(* Logix 5000 AddOnInstructionDefinition export Banner_Q2X_Param_v4; software revision 33.00 *)

TYPE Banner_IOL_Port_v4 :   // UDT that has all of the data items necessary to communicate with a specific Port on a IO-Link Master
STRUCT
   Port_Controlled : INT;   // Each bit represents a port on an IO-Link Master. Set to 1 to tell AOI to control that port.
   Port_Activate : INT;   // Each bit represents a port on an IO-Link Master. When ON that port will process any commands in queue.
   Port_Read : INT;   // Each bit represents a port on an IO-Link Master. Used to determine when device AOI has requested a Read command.
   Port_Write : INT;   // Each bit represents a port on an IO-Link Master. Used to determine when device AOI has requested a Write command.
   Port_RW_Complete : INT;   // Each bit represents a port on an IO-Link Master. Tells device AOI that Read or Write request has been completed.
   Port_Device_Read : INT;
   Data_Transfer : SINT[190];   // Array to transfer data from IO-Master to device AOIs.
END_STRUCT
END_TYPE

TYPE Banner_Q2X_BDC_v4 :   // All of the BDC data for channels 1 and 2.
STRUCT
   SP1 : DINT;   // Switchpoint.
   SP2 : DINT;   // In 2pt window mode, defines the second switching point. In other modes, SP2 is unused and must be 0.
   Switchpoint_Logic : SINT;   // 0 = Light operate, 1 = Dark operate
   BDC_Mode : SINT;   // 1 = 1pt Object Set, 128 = 2pt static BGS, 129 = 2pt Window FGS, 130 = 1pt Window FGS, 131 = Dual Mode.
   Hysteresis : INT;   // A value of 0 will result in automatically calculated hysteresis.
   Delay_Mode : SINT;   // 0 = Disabled, 1 = On Off Delay, 2 = Oneshot.
   Delay_Timer_1 : DINT;   // 0 to 90000. On delay and oneshot time.
   Delay_Timer_2 : DINT;   // 0 to 90000. Off delay only.
   Teach_Offset : SINT;   // 0 = Auto, 1 = User Selected
   FGS_Window_Size : SINT;   // 0 = Auto, 1 = User Selected
   User_Teach_Offset : DINT;   // In Object Set or Window (FGS) mode this value can be either positive or negative. In all other modes must be zero.
   FGS_User_Window_Size : DINT;   // Mode must be Window FGS. Set the +/- window value. If FGS Window Size is set to Auto this value must to set to zero.
   Auto_Thresholding : SINT;   // 0 = Slow, 1 = Medium, 2 = Fast, 3 = Off.
END_STRUCT
END_TYPE

TYPE Banner_Q2X_Pulse_Freq_v4 :
STRUCT
   Near_Freq : DINT;   // 1 to 100000 in Hz
   Far_Freq : DINT;   // 1 to 100000 in Hz
   SP1 : DINT;   // Switchpoint
   SP2 : DINT;   // In 2pt Window FGS teach, define the second switching point. In other modes SP2 should be zero.
   Pulse_Freq_LOS : DINT;   // Default value of 50. This is the Hz that the units outputs when a Loss of Signal occurs.
END_STRUCT
END_TYPE

TYPE Banner_Q2X_RD_v4 :   // UDT that stores the Write Data for a Q2X.
STRUCT
   Master_Cycle_Time : INT;
   Min_Cycle_Time : INT;
   M_Sequence_Capability : INT;
   IO_Link_Version_ID : INT;
   Process_Data_Input_Length : INT;
   Process_Data_Output_Length : INT;
   Combined_Vendor_ID : DINT;   // IO-Link Vendor ID
   Vendor_ID1 : INT;
   Vendor_ID2 : INT;
   Combined_Device_ID : DINT;   // IO-Link Device ID
   Device_ID1 : INT;
   Device_ID2 : INT;
   Device_ID3 : INT;
   Serial_Number : STRING;
   Teach_State : SINT;
   SP1_TP1 : SINT;
   SP1_TP2 : SINT;
   Measurement_1 : DINT;
   Excess_Gain : DINT;   // Amount of singla measured over the minimum threshold.
   Stability : SINT;
   Emitter_Status : SINT;   // 0 = Active, 1 = Inactive
   Temperature : DINT;
   Last_Taught_Temperature : DINT;   // Internal Temperature the last time device was taught.
   MDC_Lower_Limit : DINT;
   MDC_Upper_Limit : DINT;
   MDC_Unit : INT;
   MDC_Scale : SINT;
END_STRUCT
END_TYPE

TYPE Banner_Q2X_v4 :   // All of the parameters for a Q2X.
STRUCT
   Initial_Global_Read : BOOL;   // Determines if all of the IO-Link data has been read into the PLC yet
   Command : INT;   // Value placed in here will activate a read or write to a specifc IO-Link Index
   Read : Banner_Q2X_RD_v4;   // Read Only Data
   Write : Banner_Q2X_WD_v4;   // Write Data
   Archive : Banner_Q2X_WD_v4;   // Archive Data
   Reset : BOOL;   // Resets AOI. This will force a complete parameter read of the sensor.
END_STRUCT
END_TYPE

TYPE Banner_Q2X_WD_v4 :   // UDT that stores the Write Data for a Q2X.
STRUCT
   System_Command : INT;   // See IODD file for list of commands that can be activated via the System Command interface
   Parameter_Access_Lock : SINT;   // Write access to all parameters is prohibited while value is 1. Only this parameter can be adjusted when value is 1.
   Data_Storage_Lock : SINT;   // Automatic data storage is disabled when this value is equal to 1. Read access is not affected.
   Local_Parameterization_Lock : SINT;   // Parameterization via local control elements on device is disabled.
   Local_User_Interface_Lock : SINT;   // Operation of local user interface is disabled.
   Teach_in_Channel : SINT;   // 0 = Default, 1 = BDC1, 2 = BDC2
   Response_Speed : SINT;   // 0 = Speed 0, 1 = Speed 1, 2 = Speed 2, 3 = Speed 3
   Secondary_Output_Mode : SINT;   // 0 = Independent Output, 1 = Complementary Output, 2 = Pulse Frequency Output
   IOL_Filter_Time : INT;   // Time to average IOl process data measurement between updates
   Include_Binary : SINT;   // 0 = Include, 1 = Don't Include, 2= Measurement Device
   Measurement_1 : SINT;   // 0 = Disabled, 1 = Excess Gain, 2 = Excess Gain / 10, 3 = Channel 1 Dual Mode Percent
   Measurement_2 : SINT;   // 0 = Disabled, 1 = Distance Value, 2 = Displayed Distance, 3 = Channel 2 Dual Mode Percent
   BDC : Banner_Q2X_BDC_v4[3];
   Pulse_Freq : Banner_Q2X_Pulse_Freq_v4;
END_STRUCT
END_TYPE

ADD_ON_INSTRUCTION Banner_Q2X_Param_v4   (* revision 4.0, vendor Banner Engineering *)
// AOI to read and write parameter data to an IO-Link Q2X.
VAR_IN_OUT
   Q2X : Banner_Q2X_v4; {required}
   Port_Data : Banner_IOL_Port_v4; {required}
END_VAR
VAR_INPUT
   Port : DINT; {required}
END_VAR
VAR
   Local_Control : DINT; {access None}
   Global_Read_Command_Value : INT; {access None}
   Global_Write_Command_Value : INT; {access None}
   Command_Being_Processed : BOOL; {access None}
   Update_Archive : BOOL; {access None}
   Index_Write_Inprocess : INT; {access None}
   Index_Write_Control : INT; {access None}
   Inprocess_Index : DINT; {access None}
END_VAR

ROUTINE Logic   (* ladder *)
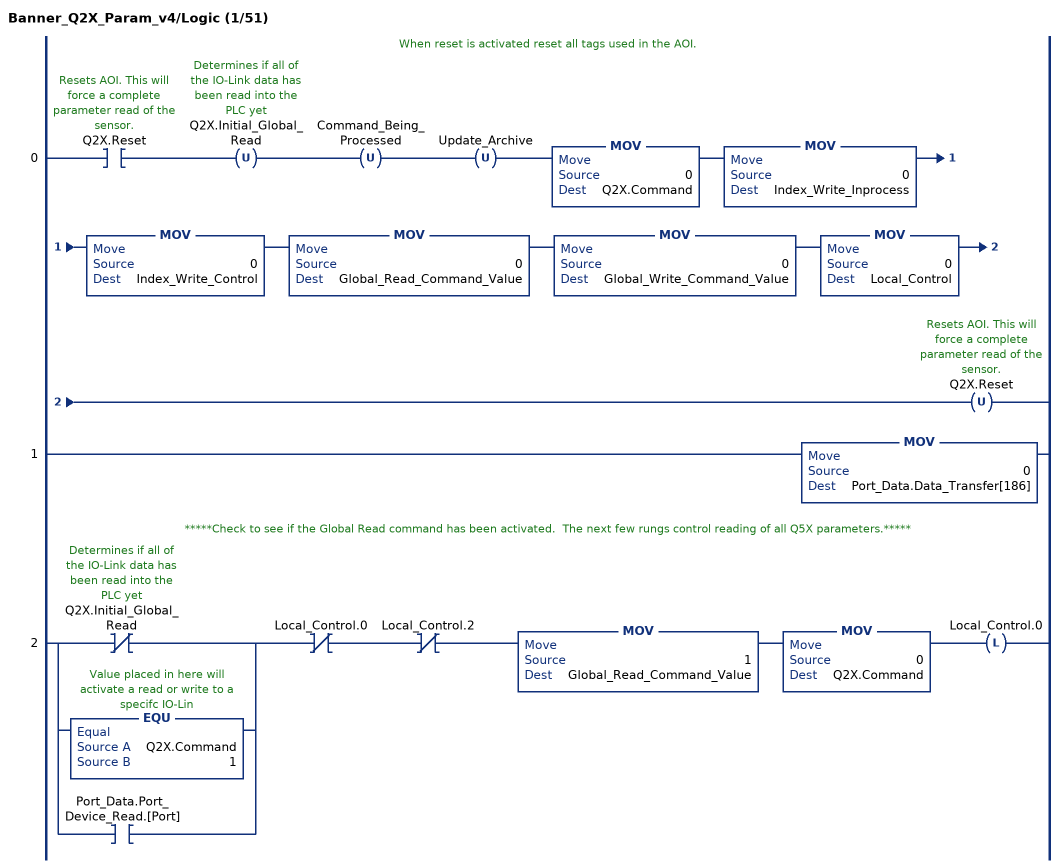
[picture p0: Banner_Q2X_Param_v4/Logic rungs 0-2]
   // When reset is activated reset all tags used in the AOI.
   0: XIC(Q2X.Reset)OTU(Q2X.Initial_Global_Read)OTU(Command_Being_Processed)OTU(Update_Archive)MOV(0,Q2X.Command)MOV(0,Index_Write_Inprocess)MOV(0,Index_Write_Control)MOV(0,Global_Read_Command_Value)MOV(0,Global_Write_Command_Value)MOV(0,Local_Control)OTU(Q2X.Reset);
   1: MOV(0,Port_Data.Data_Transfer[186]);
   // *****Check to see if the Global Read command has been activated.  The next few rungs control reading of all Q5X parameters.*****
   2: [XIO(Q2X.Initial_Global_Read) ,EQU(Q2X.Command,1) ,XIC(Port_Data.Port_Device_Read.[Port]) ]XIO(Local_Control.0)XIO(Local_Control.2)MOV(1,Global_Read_Command_Value)MOV(0,Q2X.Command)OTL(Local_Control.0);
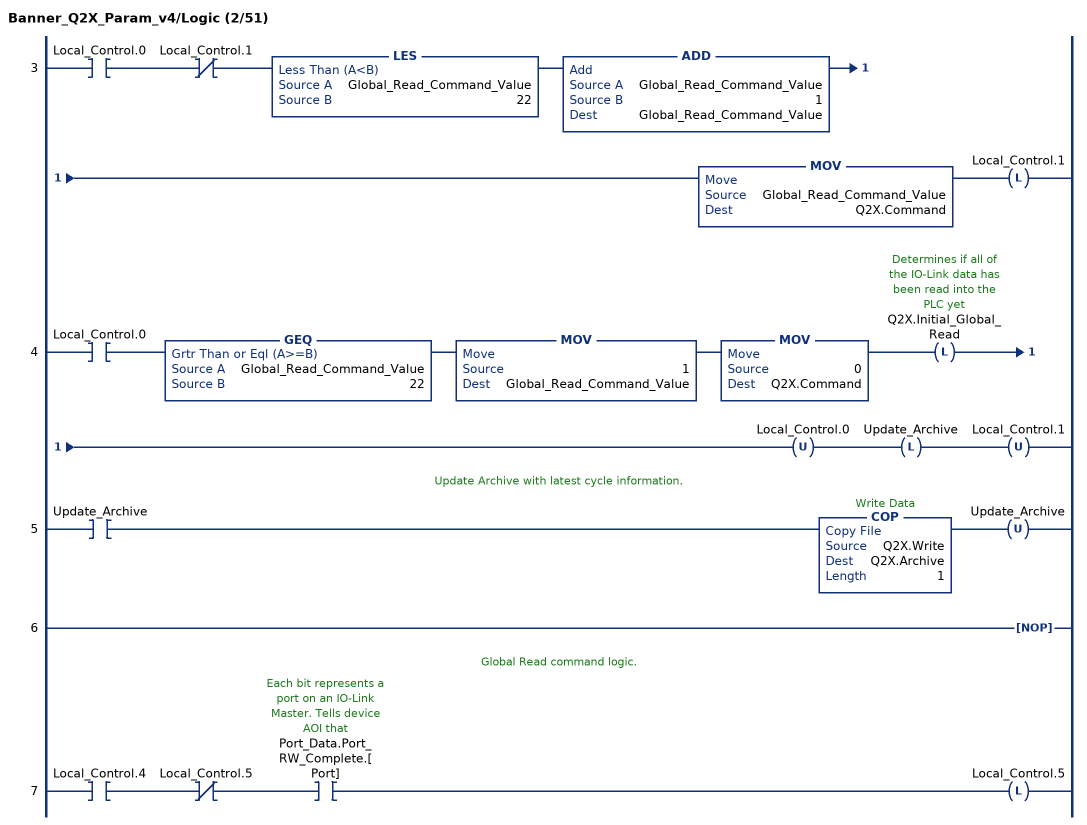
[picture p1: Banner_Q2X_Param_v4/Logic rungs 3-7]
   3: XIC(Local_Control.0)XIO(Local_Control.1)LES(Global_Read_Command_Value,22)ADD(Global_Read_Command_Value,1,Global_Read_Command_Value)MOV(Global_Read_Command_Value,Q2X.Command)OTL(Local_Control.1);
   4: XIC(Local_Control.0)GEQ(Global_Read_Command_Value,22)MOV(1,Global_Read_Command_Value)MOV(0,Q2X.Command)OTL(Q2X.Initial_Global_Read)OTU(Local_Control.0)OTL(Update_Archive)OTU(Local_Control.1);
   // Update Archive with latest cycle information.
   5: XIC(Update_Archive)COP(Q2X.Write,Q2X.Archive,1)OTU(Update_Archive);
   6: NOP();
   // Global Read command logic.
   7: XIC(Local_Control.4)XIO(Local_Control.5)XIC(Port_Data.Port_RW_Complete.[Port])OTL(Local_Control.5);
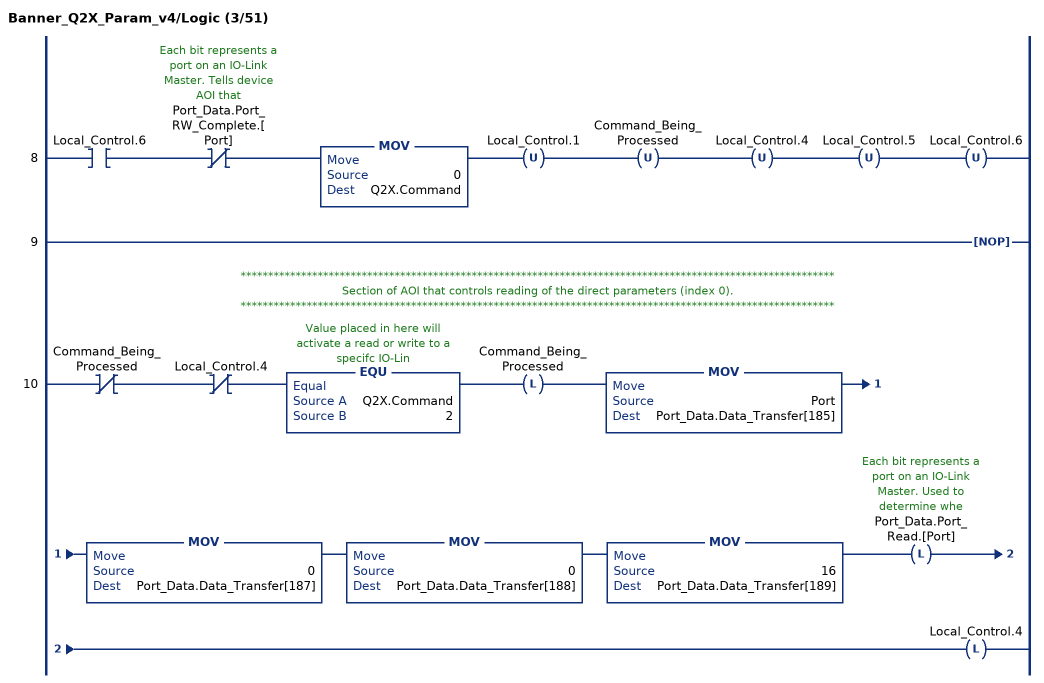
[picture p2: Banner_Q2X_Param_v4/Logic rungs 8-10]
   8: XIC(Local_Control.6)XIO(Port_Data.Port_RW_Complete.[Port])MOV(0,Q2X.Command)OTU(Local_Control.1)OTU(Command_Being_Processed)OTU(Local_Control.4)OTU(Local_Control.5)OTU(Local_Control.6);
   9: NOP();
   // ************************************************************************************************************
   // Section of AOI that controls reading of the direct parameters (index 0).
   // ************************************************************************************************************
   10: XIO(Command_Being_Processed)XIO(Local_Control.4)EQU(Q2X.Command,2)OTL(Command_Being_Processed)MOV(Port,Port_Data.Data_Transfer[185])MOV(0,Port_Data.Data_Transfer[187])MOV(0,Port_Data.Data_Transfer[188])MOV(16,Port_Data.Data_Transfer[189])OTL(Port_Data.Port_Read.[Port])OTL(Local_Control.4);
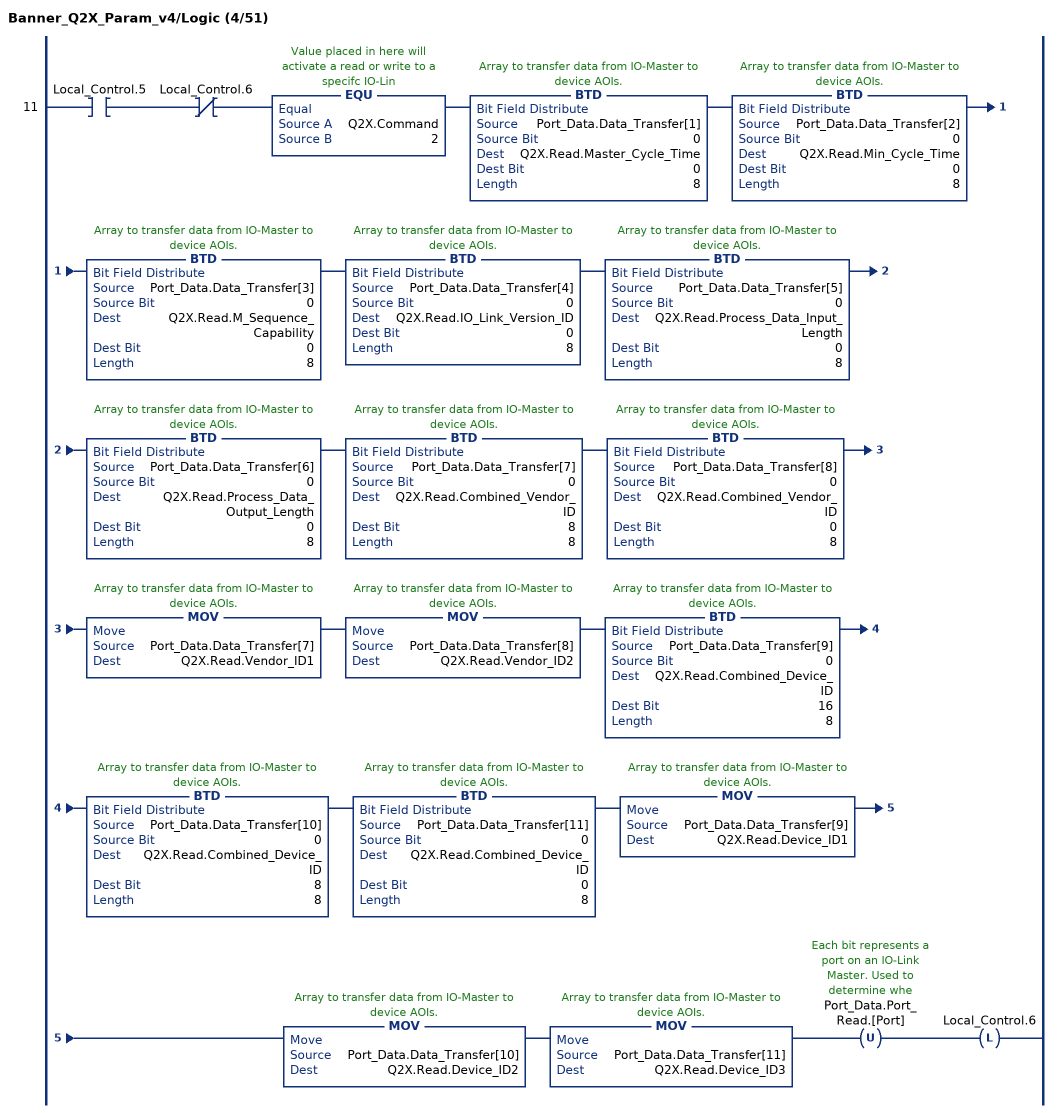
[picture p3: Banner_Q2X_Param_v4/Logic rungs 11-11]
   11: XIC(Local_Control.5)XIO(Local_Control.6)EQU(Q2X.Command,2)BTD(Port_Data.Data_Transfer[1],0,Q2X.Read.Master_Cycle_Time,0,8)BTD(Port_Data.Data_Transfer[2],0,Q2X.Read.Min_Cycle_Time,0,8)BTD(Port_Data.Data_Transfer[3],0,Q2X.Read.M_Sequence_Capability,0,8)BTD(Port_Data.Data_Transfer[4],0,Q2X.Read.IO_Link_Version_ID,0,8)BTD(Port_Data.Data_Transfer[5],0,Q2X.Read.Process_Data_Input_Length,0,8)BTD(Port_Data.Data_Transfer[6],0,Q2X.Read.Process_Data_Output_Length,0,8)BTD(Port_Data.Data_Transfer[7],0,Q2X.Read.Combined_Vendor_ID,8,8)BTD(Port_Data.Data_Transfer[8],0,Q2X.Read.Combined_Vendor_ID,0,8)MOV(Port_Data.Data_Transfer[7],Q2X.Read.Vendor_ID1)MOV(Port_Data.Data_Transfer[8],Q2X.Read.Vendor_ID2)BTD(Port_Data.Data_Transfer[9],0,Q2X.Read.Combined_Device_ID,16,8)BTD(Port_Data.Data_Transfer[10],0,Q2X.Read.Combined_Device_ID,8,8)BTD(Port_Data.Data_Transfer[11],0,Q2X.Read.Combined_Device_ID,0,8)MOV(Port_Data.Data_Transfer[9],Q2X.Read.Device_ID1)MOV(Port_Data.Data_Transfer[10],Q2X.Read.Device_ID2)MOV(Port_Data.Data_Transfer[11],Q2X.Read.Device_ID3)OTU(Port_Data.Port_Read.[Port])OTL(Local_Control.6);
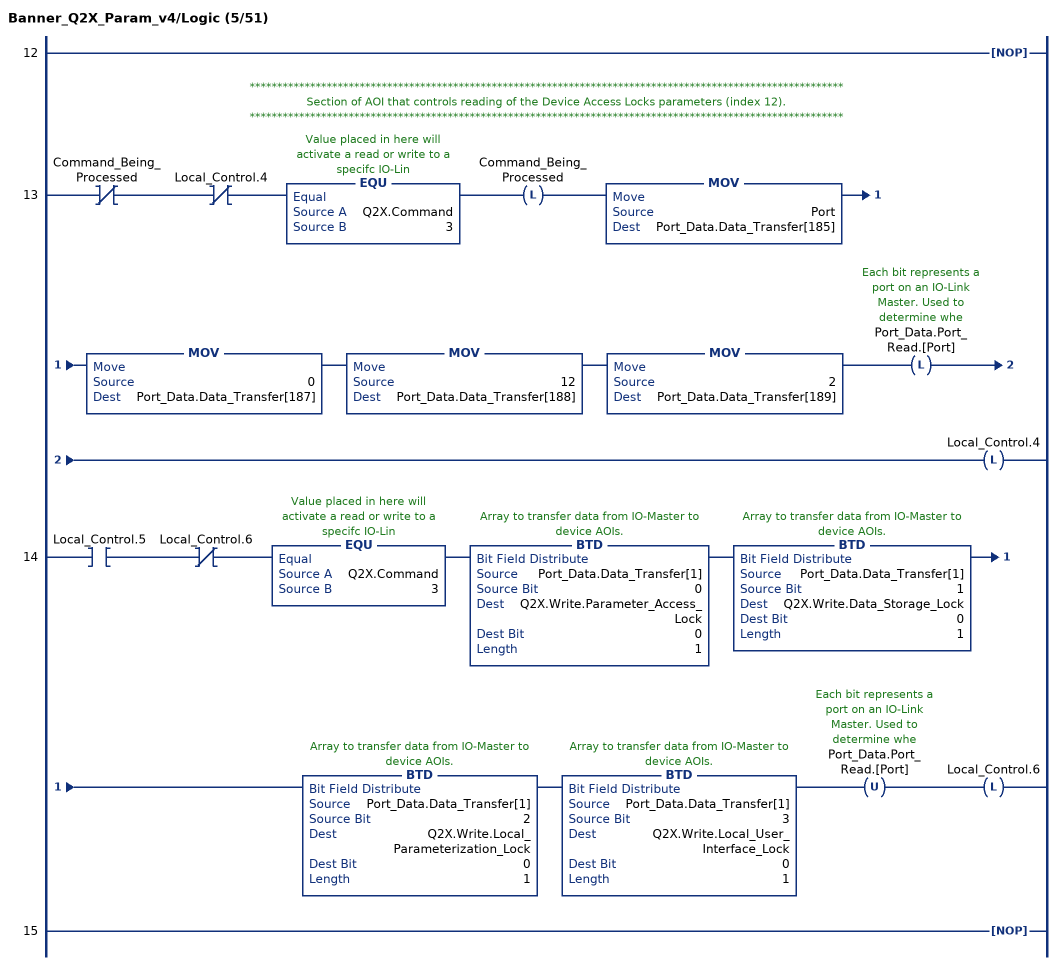
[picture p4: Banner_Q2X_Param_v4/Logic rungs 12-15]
   12: NOP();
   // ************************************************************************************************************
   // Section of AOI that controls reading of the Device Access Locks parameters (index 12).
   // ************************************************************************************************************
   13: XIO(Command_Being_Processed)XIO(Local_Control.4)EQU(Q2X.Command,3)OTL(Command_Being_Processed)MOV(Port,Port_Data.Data_Transfer[185])MOV(0,Port_Data.Data_Transfer[187])MOV(12,Port_Data.Data_Transfer[188])MOV(2,Port_Data.Data_Transfer[189])OTL(Port_Data.Port_Read.[Port])OTL(Local_Control.4);
   14: XIC(Local_Control.5)XIO(Local_Control.6)EQU(Q2X.Command,3)BTD(Port_Data.Data_Transfer[1],0,Q2X.Write.Parameter_Access_Lock,0,1)BTD(Port_Data.Data_Transfer[1],1,Q2X.Write.Data_Storage_Lock,0,1)BTD(Port_Data.Data_Transfer[1],2,Q2X.Write.Local_Parameterization_Lock,0,1)BTD(Port_Data.Data_Transfer[1],3,Q2X.Write.Local_User_Interface_Lock,0,1)OTU(Port_Data.Port_Read.[Port])OTL(Local_Control.6);
   15: NOP();
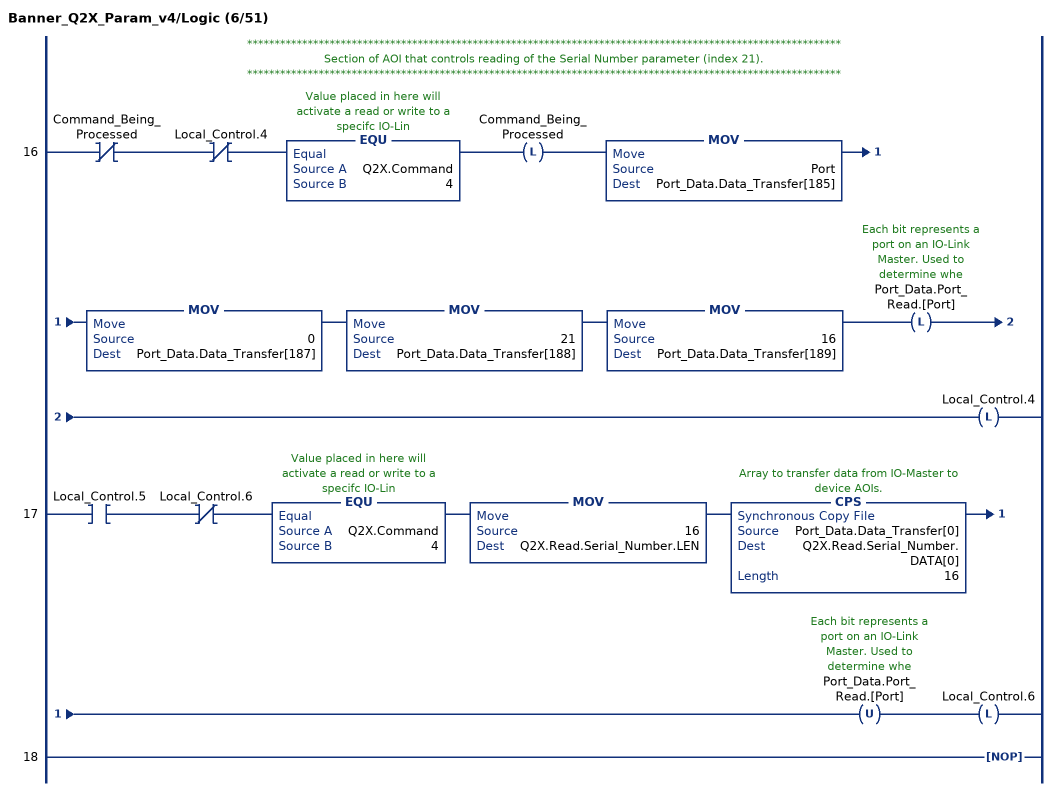
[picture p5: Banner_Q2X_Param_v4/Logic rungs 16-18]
   // ************************************************************************************************************
   // Section of AOI that controls reading of the Serial Number parameter (index 21).
   // ************************************************************************************************************
   16: XIO(Command_Being_Processed)XIO(Local_Control.4)EQU(Q2X.Command,4)OTL(Command_Being_Processed)MOV(Port,Port_Data.Data_Transfer[185])MOV(0,Port_Data.Data_Transfer[187])MOV(21,Port_Data.Data_Transfer[188])MOV(16,Port_Data.Data_Transfer[189])OTL(Port_Data.Port_Read.[Port])OTL(Local_Control.4);
   17: XIC(Local_Control.5)XIO(Local_Control.6)EQU(Q2X.Command,4)MOV(16,Q2X.Read.Serial_Number.LEN)CPS(Port_Data.Data_Transfer[0],Q2X.Read.Serial_Number.DATA[0],16)OTU(Port_Data.Port_Read.[Port])OTL(Local_Control.6);
   18: NOP();
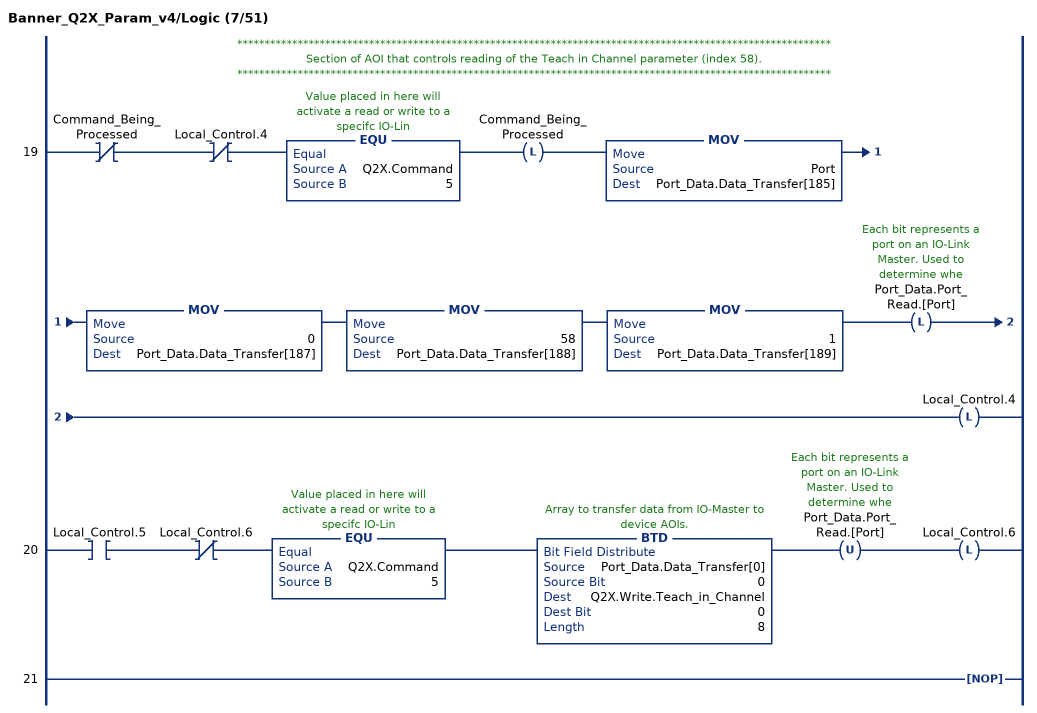
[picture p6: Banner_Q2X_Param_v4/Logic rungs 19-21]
   // ************************************************************************************************************
   // Section of AOI that controls reading of the Teach in Channel parameter (index 58).
   // ************************************************************************************************************
   19: XIO(Command_Being_Processed)XIO(Local_Control.4)EQU(Q2X.Command,5)OTL(Command_Being_Processed)MOV(Port,Port_Data.Data_Transfer[185])MOV(0,Port_Data.Data_Transfer[187])MOV(58,Port_Data.Data_Transfer[188])MOV(1,Port_Data.Data_Transfer[189])OTL(Port_Data.Port_Read.[Port])OTL(Local_Control.4);
   20: XIC(Local_Control.5)XIO(Local_Control.6)EQU(Q2X.Command,5)BTD(Port_Data.Data_Transfer[0],0,Q2X.Write.Teach_in_Channel,0,8)OTU(Port_Data.Port_Read.[Port])OTL(Local_Control.6);
   21: NOP();
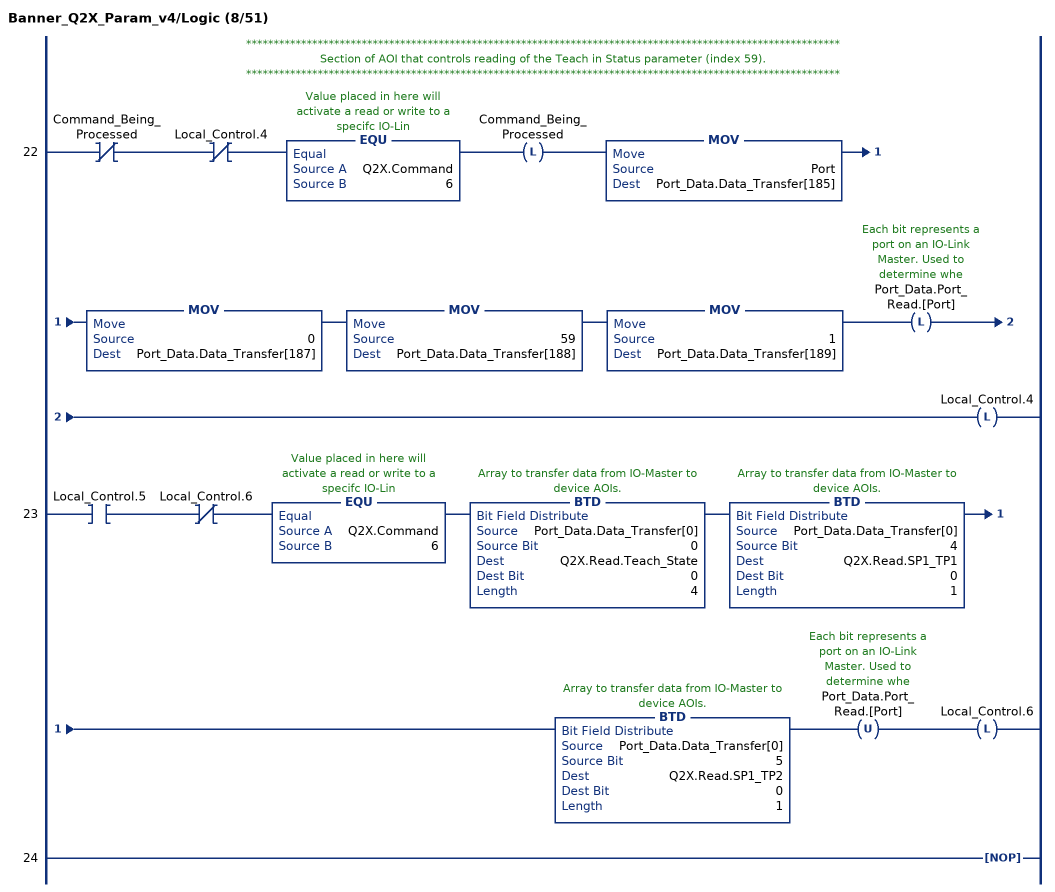
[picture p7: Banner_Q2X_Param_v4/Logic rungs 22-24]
   // ************************************************************************************************************
   // Section of AOI that controls reading of the Teach in Status parameter (index 59).
   // ************************************************************************************************************
   22: XIO(Command_Being_Processed)XIO(Local_Control.4)EQU(Q2X.Command,6)OTL(Command_Being_Processed)MOV(Port,Port_Data.Data_Transfer[185])MOV(0,Port_Data.Data_Transfer[187])MOV(59,Port_Data.Data_Transfer[188])MOV(1,Port_Data.Data_Transfer[189])OTL(Port_Data.Port_Read.[Port])OTL(Local_Control.4);
   23: XIC(Local_Control.5)XIO(Local_Control.6)EQU(Q2X.Command,6)BTD(Port_Data.Data_Transfer[0],0,Q2X.Read.Teach_State,0,4)BTD(Port_Data.Data_Transfer[0],4,Q2X.Read.SP1_TP1,0,1)BTD(Port_Data.Data_Transfer[0],5,Q2X.Read.SP1_TP2,0,1)OTU(Port_Data.Port_Read.[Port])OTL(Local_Control.6);
   24: NOP();
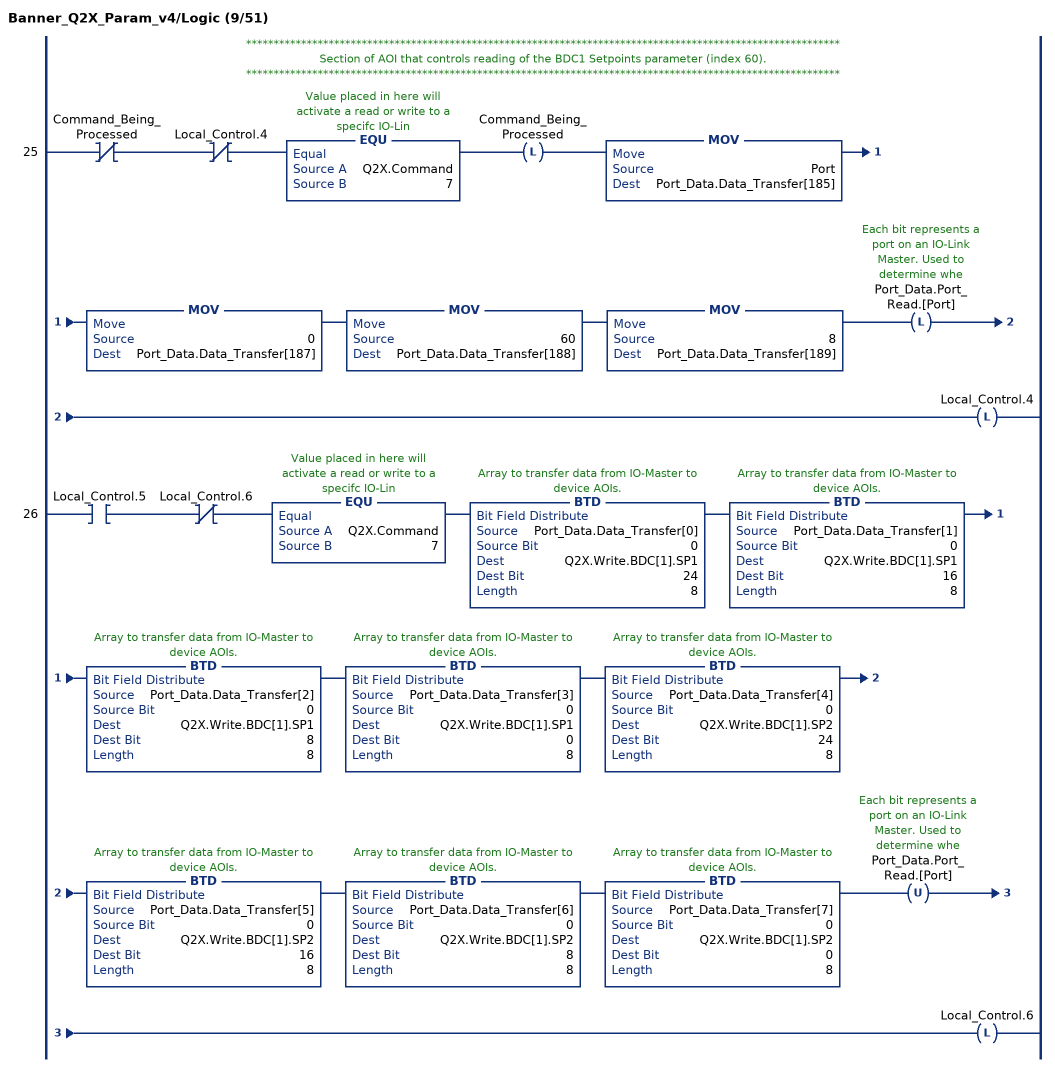
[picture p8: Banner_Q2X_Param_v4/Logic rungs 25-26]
   // ************************************************************************************************************
   // Section of AOI that controls reading of the BDC1 Setpoints parameter (index 60).
   // ************************************************************************************************************
   25: XIO(Command_Being_Processed)XIO(Local_Control.4)EQU(Q2X.Command,7)OTL(Command_Being_Processed)MOV(Port,Port_Data.Data_Transfer[185])MOV(0,Port_Data.Data_Transfer[187])MOV(60,Port_Data.Data_Transfer[188])MOV(8,Port_Data.Data_Transfer[189])OTL(Port_Data.Port_Read.[Port])OTL(Local_Control.4);
   26: XIC(Local_Control.5)XIO(Local_Control.6)EQU(Q2X.Command,7)BTD(Port_Data.Data_Transfer[0],0,Q2X.Write.BDC[1].SP1,24,8)BTD(Port_Data.Data_Transfer[1],0,Q2X.Write.BDC[1].SP1,16,8)BTD(Port_Data.Data_Transfer[2],0,Q2X.Write.BDC[1].SP1,8,8)BTD(Port_Data.Data_Transfer[3],0,Q2X.Write.BDC[1].SP1,0,8)BTD(Port_Data.Data_Transfer[4],0,Q2X.Write.BDC[1].SP2,24,8)BTD(Port_Data.Data_Transfer[5],0,Q2X.Write.BDC[1].SP2,16,8)BTD(Port_Data.Data_Transfer[6],0,Q2X.Write.BDC[1].SP2,8,8)BTD(Port_Data.Data_Transfer[7],0,Q2X.Write.BDC[1].SP2,0,8)OTU(Port_Data.Port_Read.[Port])OTL(Local_Control.6);
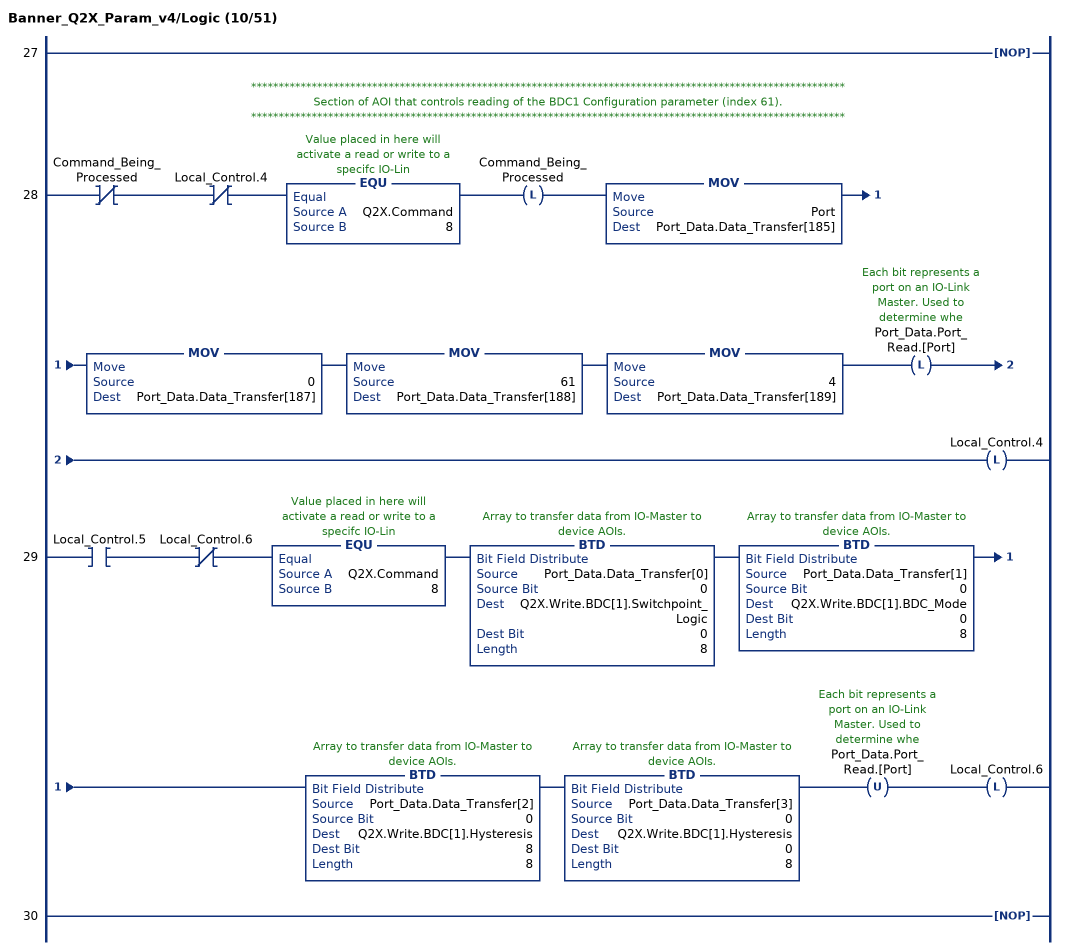
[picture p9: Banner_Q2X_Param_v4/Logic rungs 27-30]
   27: NOP();
   // ************************************************************************************************************
   // Section of AOI that controls reading of the BDC1 Configuration parameter (index 61).
   // ************************************************************************************************************
   28: XIO(Command_Being_Processed)XIO(Local_Control.4)EQU(Q2X.Command,8)OTL(Command_Being_Processed)MOV(Port,Port_Data.Data_Transfer[185])MOV(0,Port_Data.Data_Transfer[187])MOV(61,Port_Data.Data_Transfer[188])MOV(4,Port_Data.Data_Transfer[189])OTL(Port_Data.Port_Read.[Port])OTL(Local_Control.4);
   29: XIC(Local_Control.5)XIO(Local_Control.6)EQU(Q2X.Command,8)BTD(Port_Data.Data_Transfer[0],0,Q2X.Write.BDC[1].Switchpoint_Logic,0,8)BTD(Port_Data.Data_Transfer[1],0,Q2X.Write.BDC[1].BDC_Mode,0,8)BTD(Port_Data.Data_Transfer[2],0,Q2X.Write.BDC[1].Hysteresis,8,8)BTD(Port_Data.Data_Transfer[3],0,Q2X.Write.BDC[1].Hysteresis,0,8)OTU(Port_Data.Port_Read.[Port])OTL(Local_Control.6);
   30: NOP();
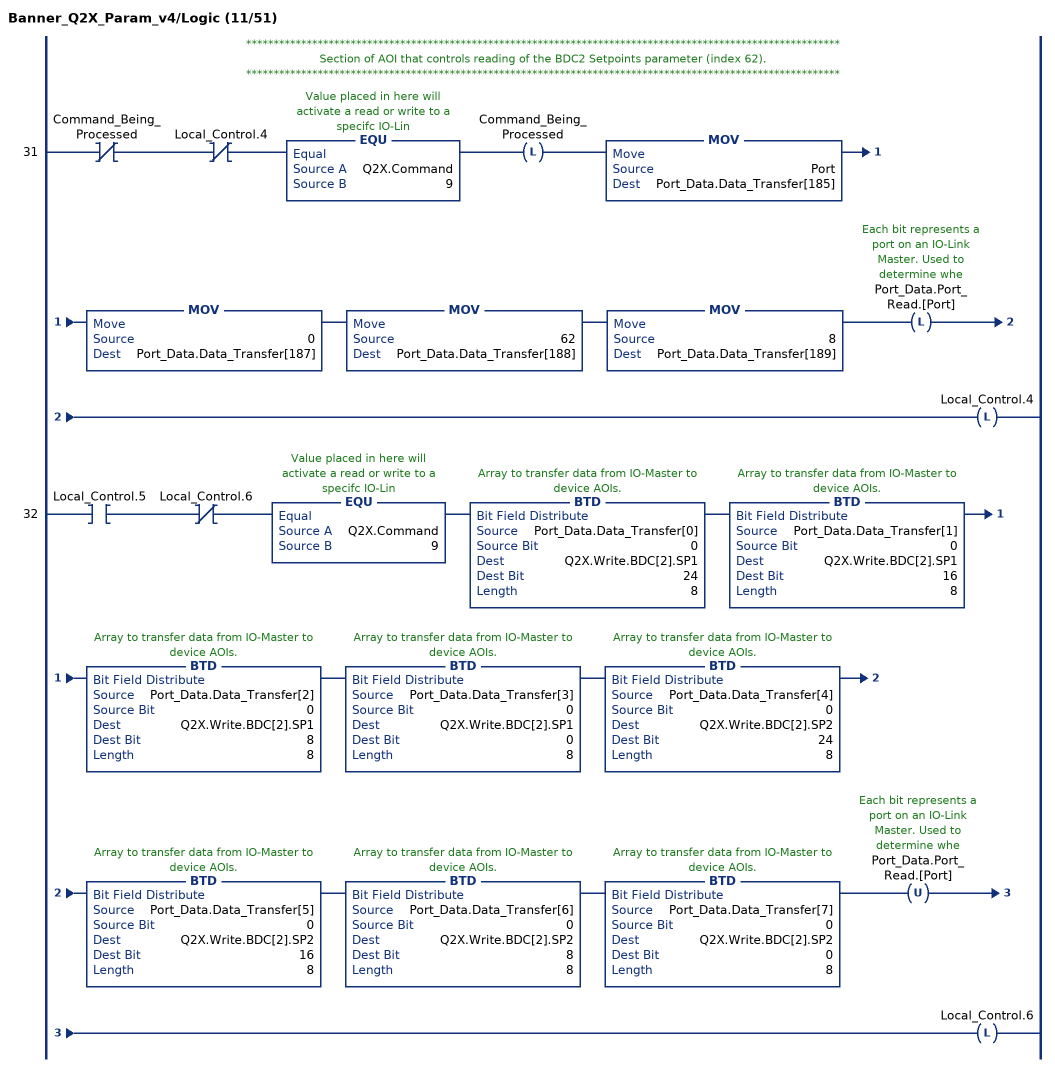
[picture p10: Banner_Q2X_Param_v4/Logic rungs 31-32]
   // ************************************************************************************************************
   // Section of AOI that controls reading of the BDC2 Setpoints parameter (index 62).
   // ************************************************************************************************************
   31: XIO(Command_Being_Processed)XIO(Local_Control.4)EQU(Q2X.Command,9)OTL(Command_Being_Processed)MOV(Port,Port_Data.Data_Transfer[185])MOV(0,Port_Data.Data_Transfer[187])MOV(62,Port_Data.Data_Transfer[188])MOV(8,Port_Data.Data_Transfer[189])OTL(Port_Data.Port_Read.[Port])OTL(Local_Control.4);
   32: XIC(Local_Control.5)XIO(Local_Control.6)EQU(Q2X.Command,9)BTD(Port_Data.Data_Transfer[0],0,Q2X.Write.BDC[2].SP1,24,8)BTD(Port_Data.Data_Transfer[1],0,Q2X.Write.BDC[2].SP1,16,8)BTD(Port_Data.Data_Transfer[2],0,Q2X.Write.BDC[2].SP1,8,8)BTD(Port_Data.Data_Transfer[3],0,Q2X.Write.BDC[2].SP1,0,8)BTD(Port_Data.Data_Transfer[4],0,Q2X.Write.BDC[2].SP2,24,8)BTD(Port_Data.Data_Transfer[5],0,Q2X.Write.BDC[2].SP2,16,8)BTD(Port_Data.Data_Transfer[6],0,Q2X.Write.BDC[2].SP2,8,8)BTD(Port_Data.Data_Transfer[7],0,Q2X.Write.BDC[2].SP2,0,8)OTU(Port_Data.Port_Read.[Port])OTL(Local_Control.6);
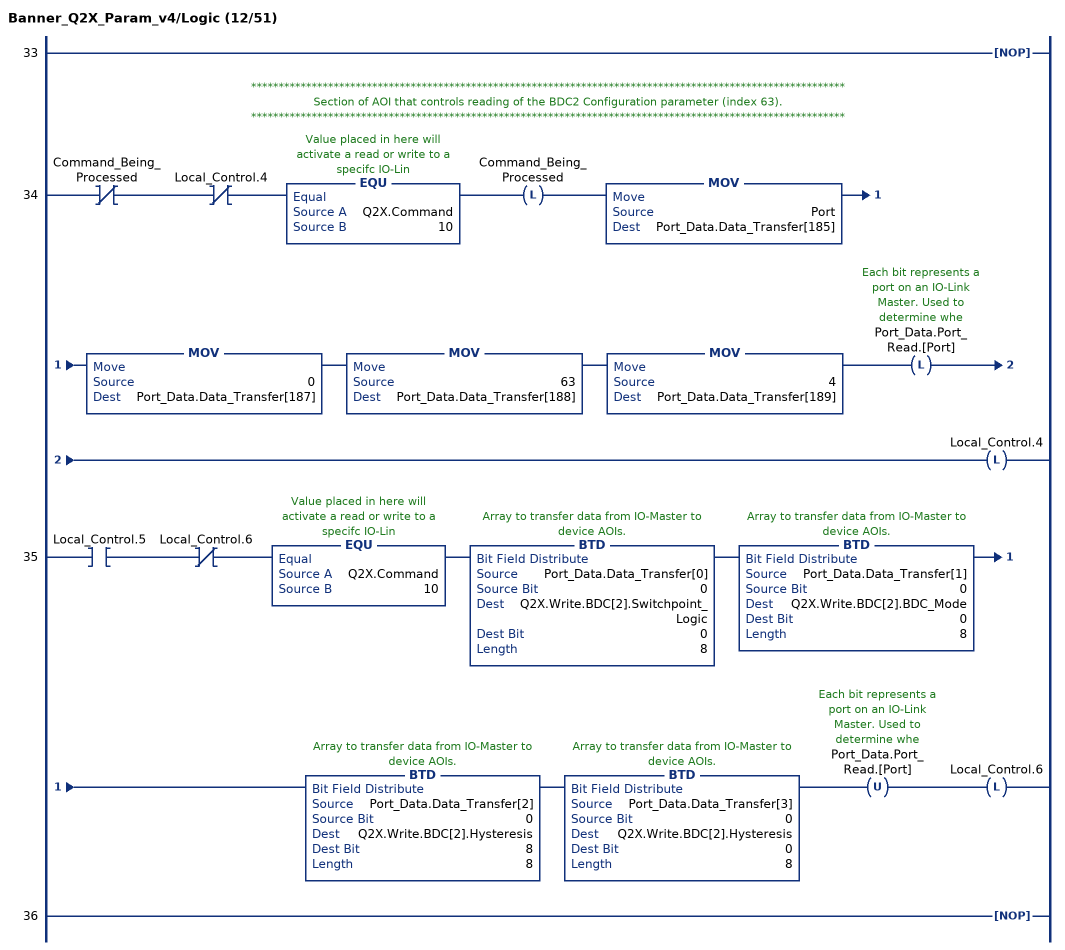
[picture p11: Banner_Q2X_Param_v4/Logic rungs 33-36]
   33: NOP();
   // ************************************************************************************************************
   // Section of AOI that controls reading of the BDC2 Configuration parameter (index 63).
   // ************************************************************************************************************
   34: XIO(Command_Being_Processed)XIO(Local_Control.4)EQU(Q2X.Command,10)OTL(Command_Being_Processed)MOV(Port,Port_Data.Data_Transfer[185])MOV(0,Port_Data.Data_Transfer[187])MOV(63,Port_Data.Data_Transfer[188])MOV(4,Port_Data.Data_Transfer[189])OTL(Port_Data.Port_Read.[Port])OTL(Local_Control.4);
   35: XIC(Local_Control.5)XIO(Local_Control.6)EQU(Q2X.Command,10)BTD(Port_Data.Data_Transfer[0],0,Q2X.Write.BDC[2].Switchpoint_Logic,0,8)BTD(Port_Data.Data_Transfer[1],0,Q2X.Write.BDC[2].BDC_Mode,0,8)BTD(Port_Data.Data_Transfer[2],0,Q2X.Write.BDC[2].Hysteresis,8,8)BTD(Port_Data.Data_Transfer[3],0,Q2X.Write.BDC[2].Hysteresis,0,8)OTU(Port_Data.Port_Read.[Port])OTL(Local_Control.6);
   36: NOP();
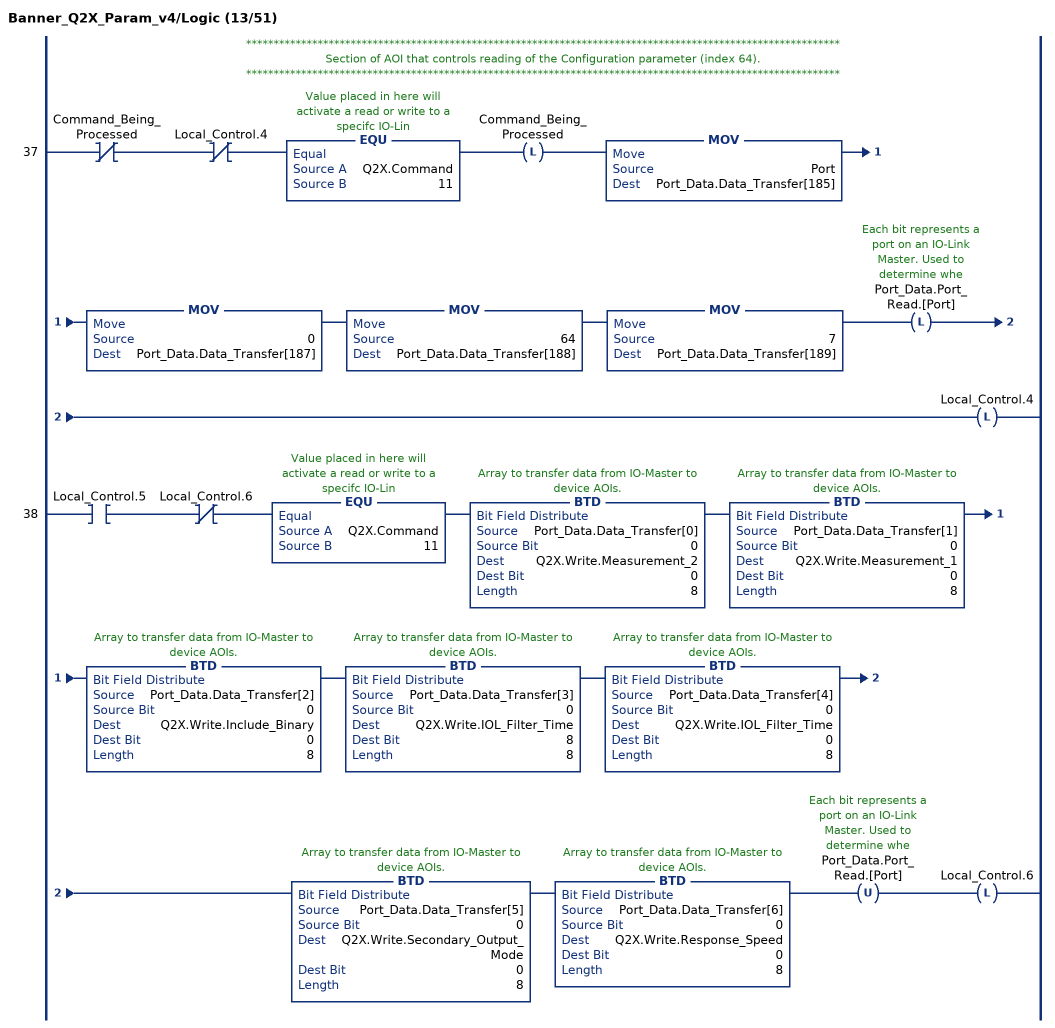
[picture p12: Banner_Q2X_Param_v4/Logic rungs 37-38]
   // ************************************************************************************************************
   // Section of AOI that controls reading of the Configuration parameter (index 64).
   // ************************************************************************************************************
   37: XIO(Command_Being_Processed)XIO(Local_Control.4)EQU(Q2X.Command,11)OTL(Command_Being_Processed)MOV(Port,Port_Data.Data_Transfer[185])MOV(0,Port_Data.Data_Transfer[187])MOV(64,Port_Data.Data_Transfer[188])MOV(7,Port_Data.Data_Transfer[189])OTL(Port_Data.Port_Read.[Port])OTL(Local_Control.4);
   38: XIC(Local_Control.5)XIO(Local_Control.6)EQU(Q2X.Command,11)BTD(Port_Data.Data_Transfer[0],0,Q2X.Write.Measurement_2,0,8)BTD(Port_Data.Data_Transfer[1],0,Q2X.Write.Measurement_1,0,8)BTD(Port_Data.Data_Transfer[2],0,Q2X.Write.Include_Binary,0,8)BTD(Port_Data.Data_Transfer[3],0,Q2X.Write.IOL_Filter_Time,8,8)BTD(Port_Data.Data_Transfer[4],0,Q2X.Write.IOL_Filter_Time,0,8)BTD(Port_Data.Data_Transfer[5],0,Q2X.Write.Secondary_Output_Mode,0,8)BTD(Port_Data.Data_Transfer[6],0,Q2X.Write.Response_Speed,0,8)OTU(Port_Data.Port_Read.[Port])OTL(Local_Control.6);
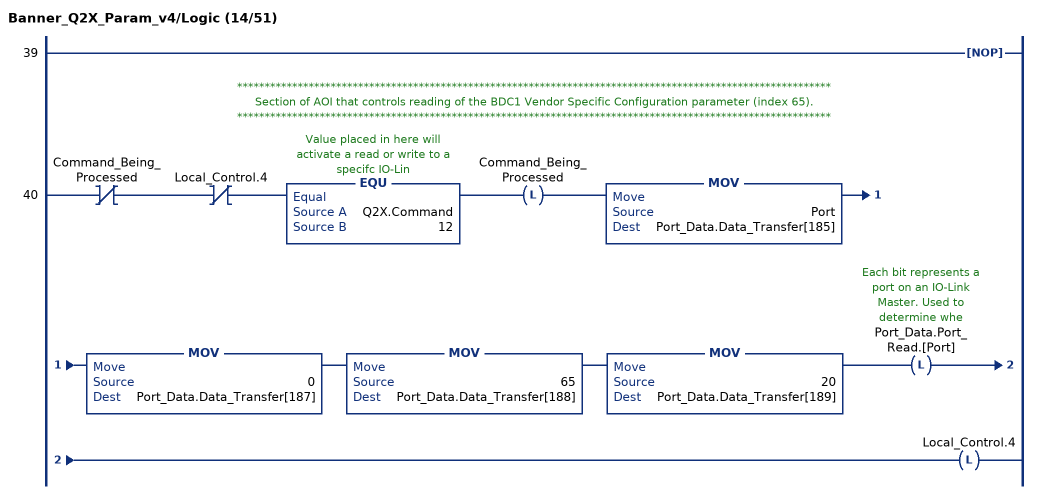
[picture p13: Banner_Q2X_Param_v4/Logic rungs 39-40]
   39: NOP();
   // ************************************************************************************************************
   // Section of AOI that controls reading of the BDC1 Vendor Specific Configuration parameter (index 65).
   // ************************************************************************************************************
   40: XIO(Command_Being_Processed)XIO(Local_Control.4)EQU(Q2X.Command,12)OTL(Command_Being_Processed)MOV(Port,Port_Data.Data_Transfer[185])MOV(0,Port_Data.Data_Transfer[187])MOV(65,Port_Data.Data_Transfer[188])MOV(20,Port_Data.Data_Transfer[189])OTL(Port_Data.Port_Read.[Port])OTL(Local_Control.4);
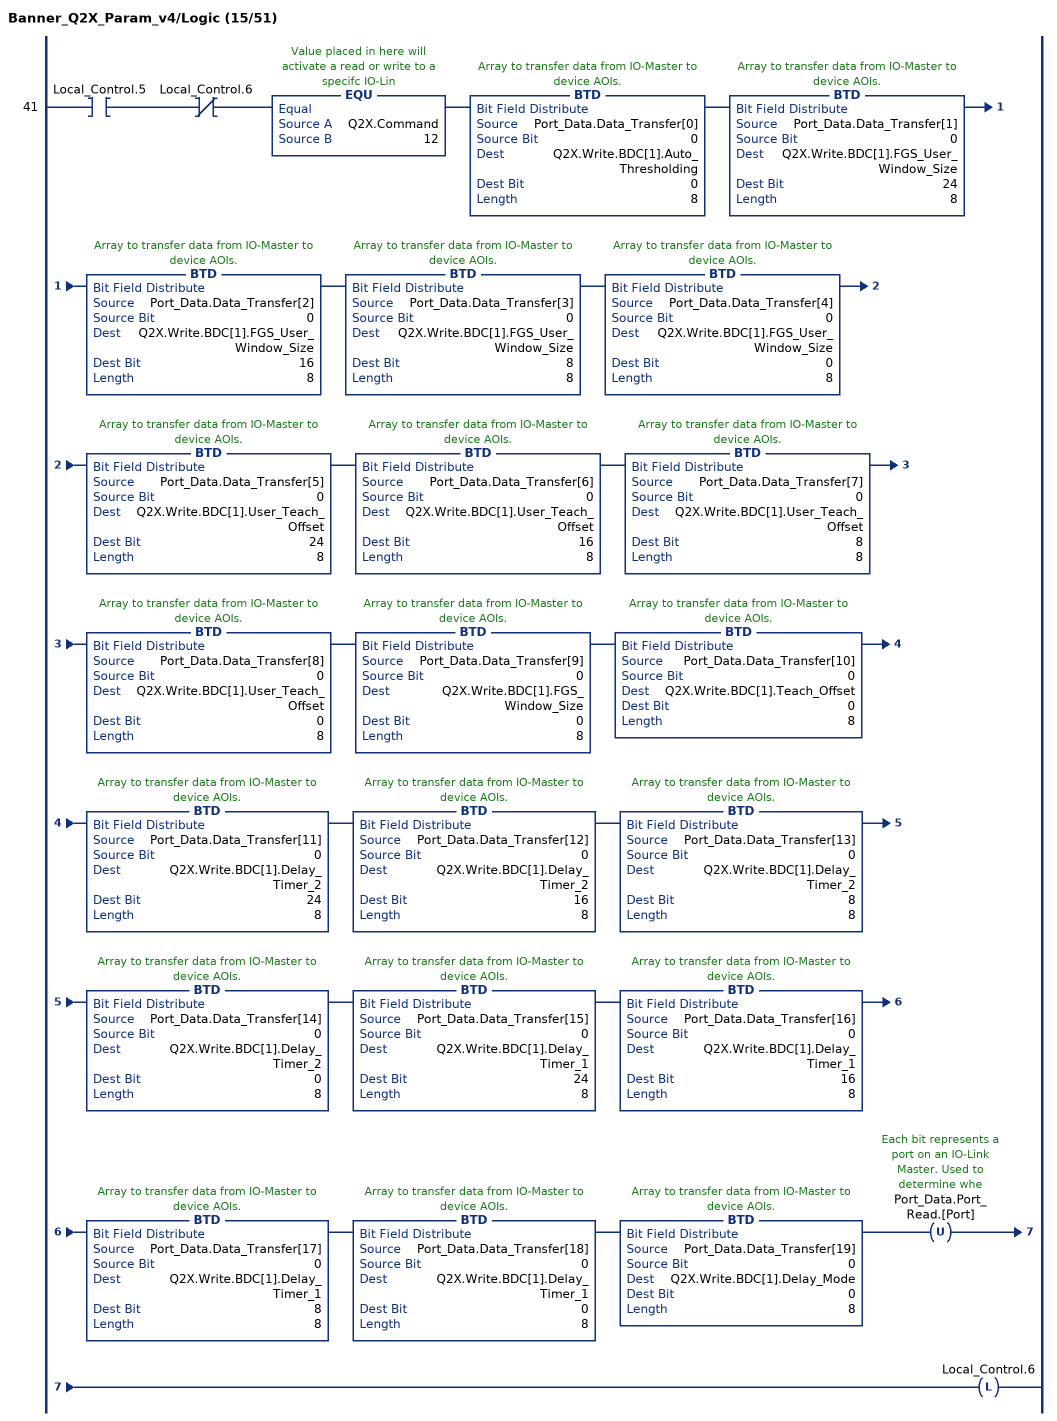
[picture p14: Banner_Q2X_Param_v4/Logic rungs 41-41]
   41: XIC(Local_Control.5)XIO(Local_Control.6)EQU(Q2X.Command,12)BTD(Port_Data.Data_Transfer[0],0,Q2X.Write.BDC[1].Auto_Thresholding,0,8)BTD(Port_Data.Data_Transfer[1],0,Q2X.Write.BDC[1].FGS_User_Window_Size,24,8)BTD(Port_Data.Data_Transfer[2],0,Q2X.Write.BDC[1].FGS_User_Window_Size,16,8)BTD(Port_Data.Data_Transfer[3],0,Q2X.Write.BDC[1].FGS_User_Window_Size,8,8)BTD(Port_Data.Data_Transfer[4],0,Q2X.Write.BDC[1].FGS_User_Window_Size,0,8)BTD(Port_Data.Data_Transfer[5],0,Q2X.Write.BDC[1].User_Teach_Offset,24,8)BTD(Port_Data.Data_Transfer[6],0,Q2X.Write.BDC[1].User_Teach_Offset,16,8)BTD(Port_Data.Data_Transfer[7],0,Q2X.Write.BDC[1].User_Teach_Offset,8,8)BTD(Port_Data.Data_Transfer[8],0,Q2X.Write.BDC[1].User_Teach_Offset,0,8)BTD(Port_Data.Data_Transfer[9],0,Q2X.Write.BDC[1].FGS_Window_Size,0,8)BTD(Port_Data.Data_Transfer[10],0,Q2X.Write.BDC[1].Teach_Offset,0,8)BTD(Port_Data.Data_Transfer[11],0,Q2X.Write.BDC[1].Delay_Timer_2,24,8)BTD(Port_Data.Data_Transfer[12],0,Q2X.Write.BDC[1].Delay_Timer_2,16,8)BTD(Port_Data.Data_Transfer[13],0,Q2X.Write.BDC[1].Delay_Timer_2,8,8)BTD(Port_Data.Data_Transfer[14],0,Q2X.Write.BDC[1].Delay_Timer_2,0,8)BTD(Port_Data.Data_Transfer[15],0,Q2X.Write.BDC[1].Delay_Timer_1,24,8)BTD(Port_Data.Data_Transfer[16],0,Q2X.Write.BDC[1].Delay_Timer_1,16,8)BTD(Port_Data.Data_Transfer[17],0,Q2X.Write.BDC[1].Delay_Timer_1,8,8)BTD(Port_Data.Data_Transfer[18],0,Q2X.Write.BDC[1].Delay_Timer_1,0,8)BTD(Port_Data.Data_Transfer[19],0,Q2X.Write.BDC[1].Delay_Mode,0,8)OTU(Port_Data.Port_Read.[Port])OTL(Local_Control.6);
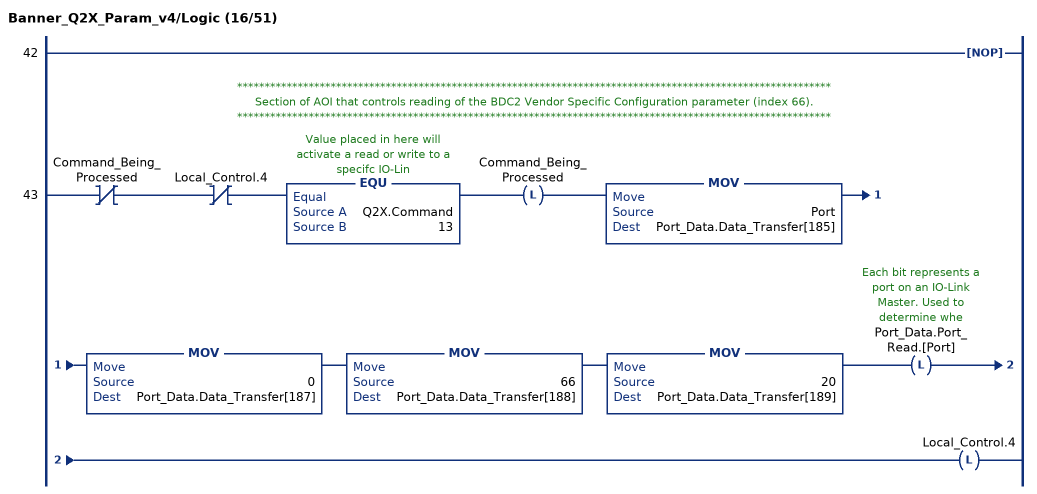
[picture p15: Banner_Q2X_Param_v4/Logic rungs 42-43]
   42: NOP();
   // ************************************************************************************************************
   // Section of AOI that controls reading of the BDC2 Vendor Specific Configuration parameter (index 66).
   // ************************************************************************************************************
   43: XIO(Command_Being_Processed)XIO(Local_Control.4)EQU(Q2X.Command,13)OTL(Command_Being_Processed)MOV(Port,Port_Data.Data_Transfer[185])MOV(0,Port_Data.Data_Transfer[187])MOV(66,Port_Data.Data_Transfer[188])MOV(20,Port_Data.Data_Transfer[189])OTL(Port_Data.Port_Read.[Port])OTL(Local_Control.4);
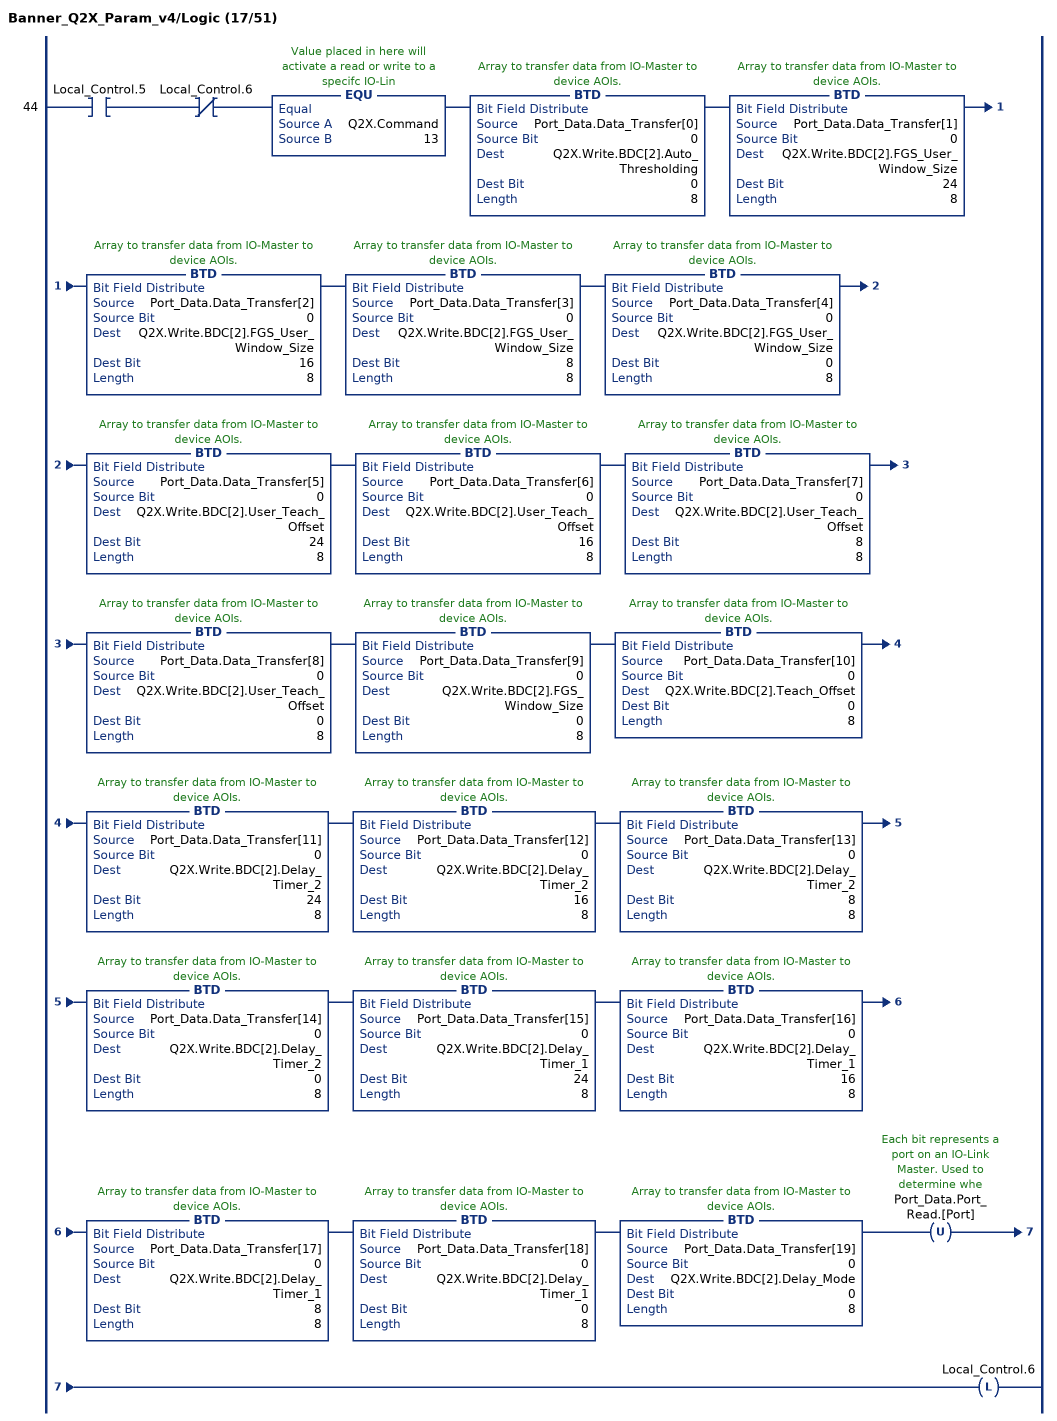
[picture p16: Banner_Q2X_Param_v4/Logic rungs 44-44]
   44: XIC(Local_Control.5)XIO(Local_Control.6)EQU(Q2X.Command,13)BTD(Port_Data.Data_Transfer[0],0,Q2X.Write.BDC[2].Auto_Thresholding,0,8)BTD(Port_Data.Data_Transfer[1],0,Q2X.Write.BDC[2].FGS_User_Window_Size,24,8)BTD(Port_Data.Data_Transfer[2],0,Q2X.Write.BDC[2].FGS_User_Window_Size,16,8)BTD(Port_Data.Data_Transfer[3],0,Q2X.Write.BDC[2].FGS_User_Window_Size,8,8)BTD(Port_Data.Data_Transfer[4],0,Q2X.Write.BDC[2].FGS_User_Window_Size,0,8)BTD(Port_Data.Data_Transfer[5],0,Q2X.Write.BDC[2].User_Teach_Offset,24,8)BTD(Port_Data.Data_Transfer[6],0,Q2X.Write.BDC[2].User_Teach_Offset,16,8)BTD(Port_Data.Data_Transfer[7],0,Q2X.Write.BDC[2].User_Teach_Offset,8,8)BTD(Port_Data.Data_Transfer[8],0,Q2X.Write.BDC[2].User_Teach_Offset,0,8)BTD(Port_Data.Data_Transfer[9],0,Q2X.Write.BDC[2].FGS_Window_Size,0,8)BTD(Port_Data.Data_Transfer[10],0,Q2X.Write.BDC[2].Teach_Offset,0,8)BTD(Port_Data.Data_Transfer[11],0,Q2X.Write.BDC[2].Delay_Timer_2,24,8)BTD(Port_Data.Data_Transfer[12],0,Q2X.Write.BDC[2].Delay_Timer_2,16,8)BTD(Port_Data.Data_Transfer[13],0,Q2X.Write.BDC[2].Delay_Timer_2,8,8)BTD(Port_Data.Data_Transfer[14],0,Q2X.Write.BDC[2].Delay_Timer_2,0,8)BTD(Port_Data.Data_Transfer[15],0,Q2X.Write.BDC[2].Delay_Timer_1,24,8)BTD(Port_Data.Data_Transfer[16],0,Q2X.Write.BDC[2].Delay_Timer_1,16,8)BTD(Port_Data.Data_Transfer[17],0,Q2X.Write.BDC[2].Delay_Timer_1,8,8)BTD(Port_Data.Data_Transfer[18],0,Q2X.Write.BDC[2].Delay_Timer_1,0,8)BTD(Port_Data.Data_Transfer[19],0,Q2X.Write.BDC[2].Delay_Mode,0,8)OTU(Port_Data.Port_Read.[Port])OTL(Local_Control.6);
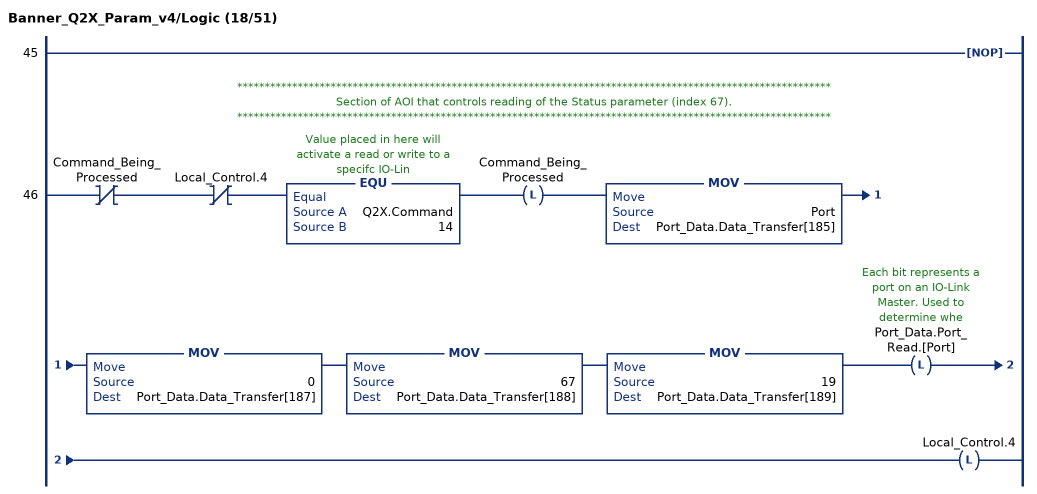
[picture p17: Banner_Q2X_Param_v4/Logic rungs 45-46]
   45: NOP();
   // ************************************************************************************************************
   // Section of AOI that controls reading of the Status parameter (index 67).
   // ************************************************************************************************************
   46: XIO(Command_Being_Processed)XIO(Local_Control.4)EQU(Q2X.Command,14)OTL(Command_Being_Processed)MOV(Port,Port_Data.Data_Transfer[185])MOV(0,Port_Data.Data_Transfer[187])MOV(67,Port_Data.Data_Transfer[188])MOV(19,Port_Data.Data_Transfer[189])OTL(Port_Data.Port_Read.[Port])OTL(Local_Control.4);
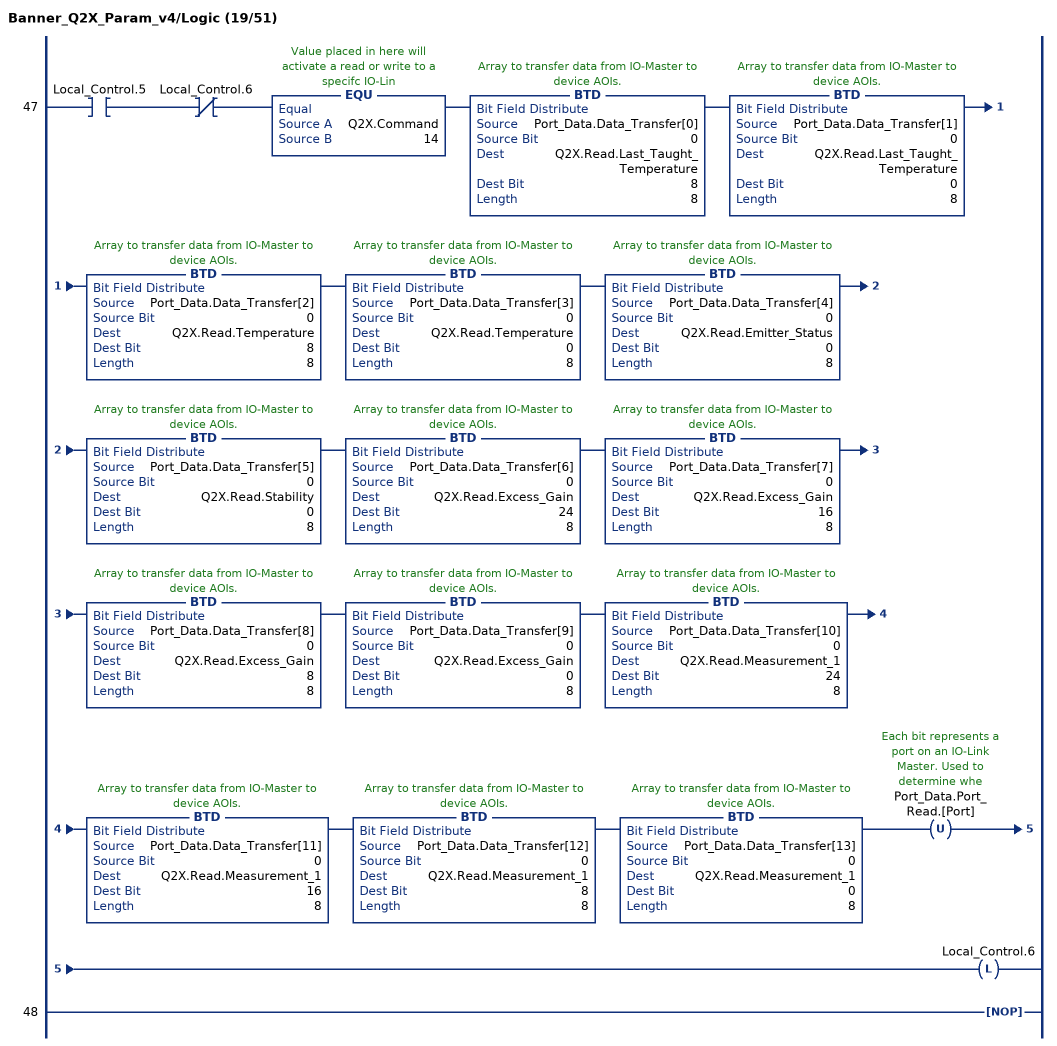
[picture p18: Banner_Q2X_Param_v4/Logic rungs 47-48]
   47: XIC(Local_Control.5)XIO(Local_Control.6)EQU(Q2X.Command,14)BTD(Port_Data.Data_Transfer[0],0,Q2X.Read.Last_Taught_Temperature,8,8)BTD(Port_Data.Data_Transfer[1],0,Q2X.Read.Last_Taught_Temperature,0,8)BTD(Port_Data.Data_Transfer[2],0,Q2X.Read.Temperature,8,8)BTD(Port_Data.Data_Transfer[3],0,Q2X.Read.Temperature,0,8)BTD(Port_Data.Data_Transfer[4],0,Q2X.Read.Emitter_Status,0,8)BTD(Port_Data.Data_Transfer[5],0,Q2X.Read.Stability,0,8)BTD(Port_Data.Data_Transfer[6],0,Q2X.Read.Excess_Gain,24,8)BTD(Port_Data.Data_Transfer[7],0,Q2X.Read.Excess_Gain,16,8)BTD(Port_Data.Data_Transfer[8],0,Q2X.Read.Excess_Gain,8,8)BTD(Port_Data.Data_Transfer[9],0,Q2X.Read.Excess_Gain,0,8)BTD(Port_Data.Data_Transfer[10],0,Q2X.Read.Measurement_1,24,8)BTD(Port_Data.Data_Transfer[11],0,Q2X.Read.Measurement_1,16,8)BTD(Port_Data.Data_Transfer[12],0,Q2X.Read.Measurement_1,8,8)BTD(Port_Data.Data_Transfer[13],0,Q2X.Read.Measurement_1,0,8)OTU(Port_Data.Port_Read.[Port])OTL(Local_Control.6);
   48: NOP();
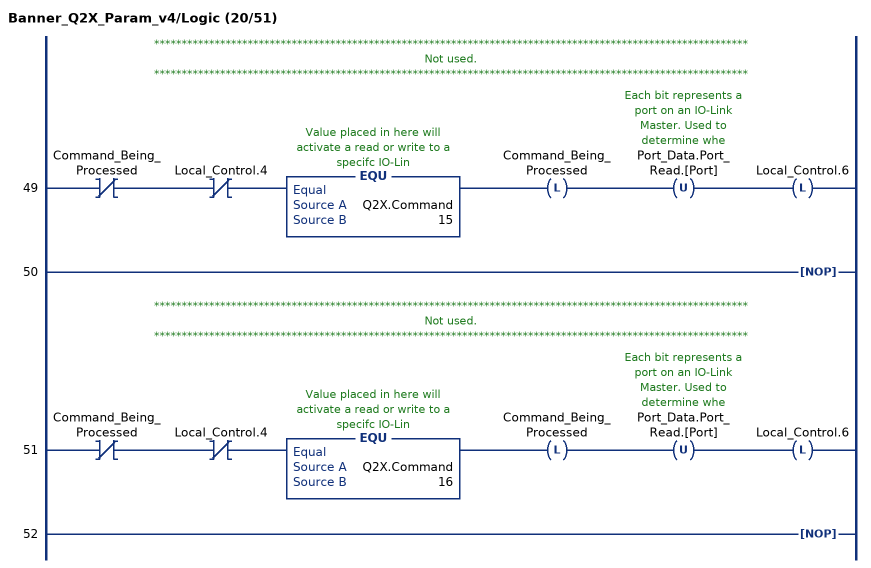
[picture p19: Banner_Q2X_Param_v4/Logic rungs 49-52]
   // ************************************************************************************************************
   // Not used.
   // ************************************************************************************************************
   49: XIO(Command_Being_Processed)XIO(Local_Control.4)EQU(Q2X.Command,15)OTL(Command_Being_Processed)OTU(Port_Data.Port_Read.[Port])OTL(Local_Control.6);
   50: NOP();
   // ************************************************************************************************************
   // Not used.
   // ************************************************************************************************************
   51: XIO(Command_Being_Processed)XIO(Local_Control.4)EQU(Q2X.Command,16)OTL(Command_Being_Processed)OTU(Port_Data.Port_Read.[Port])OTL(Local_Control.6);
   52: NOP();
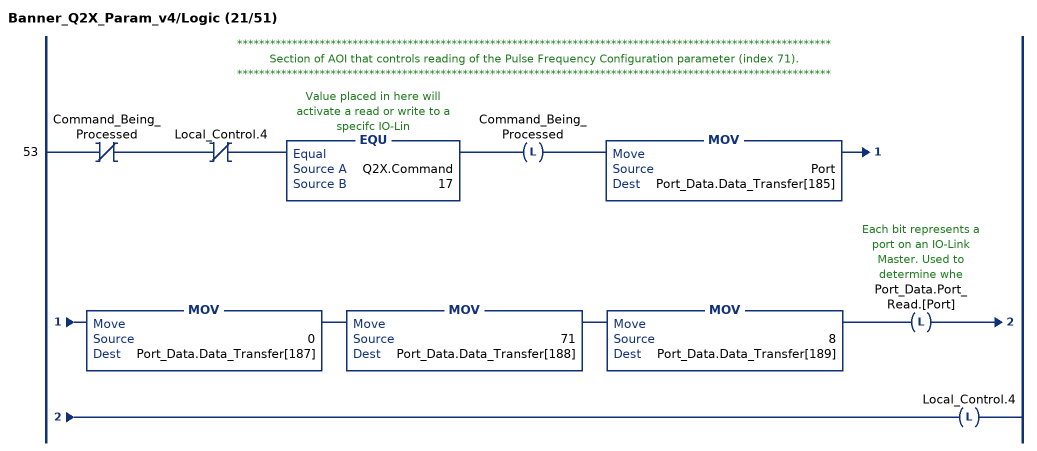
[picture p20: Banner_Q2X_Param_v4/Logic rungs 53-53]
   // ************************************************************************************************************
   // Section of AOI that controls reading of the Pulse Frequency Configuration parameter (index 71).
   // ************************************************************************************************************
   53: XIO(Command_Being_Processed)XIO(Local_Control.4)EQU(Q2X.Command,17)OTL(Command_Being_Processed)MOV(Port,Port_Data.Data_Transfer[185])MOV(0,Port_Data.Data_Transfer[187])MOV(71,Port_Data.Data_Transfer[188])MOV(8,Port_Data.Data_Transfer[189])OTL(Port_Data.Port_Read.[Port])OTL(Local_Control.4);
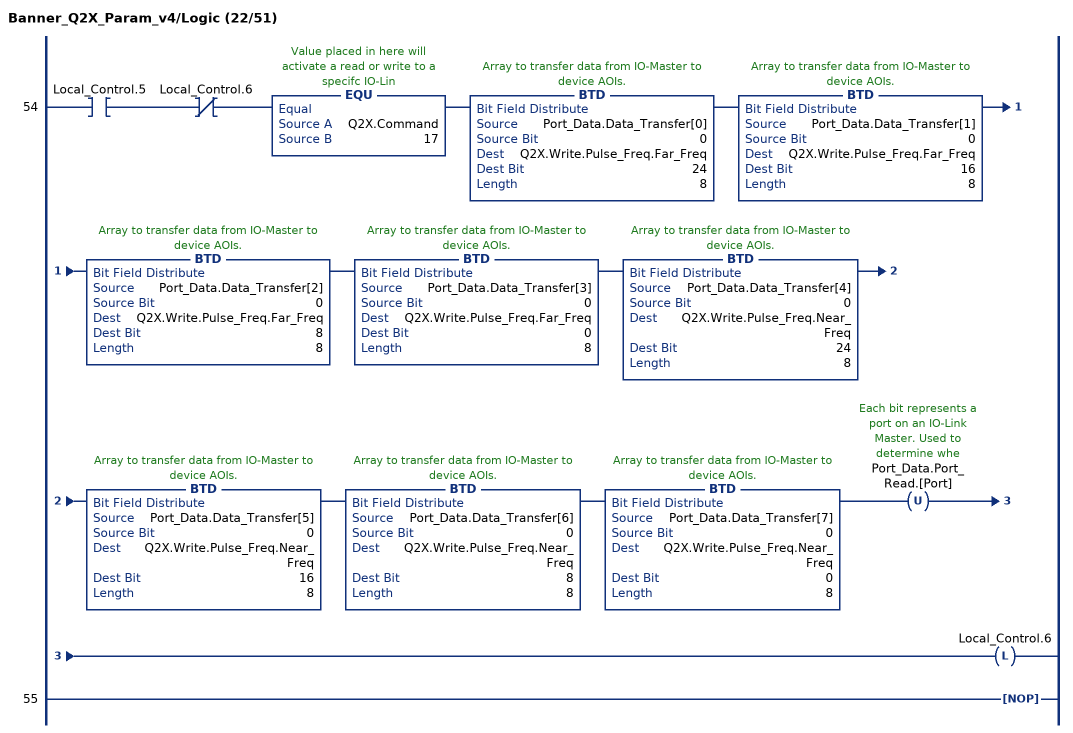
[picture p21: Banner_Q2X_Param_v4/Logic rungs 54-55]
   54: XIC(Local_Control.5)XIO(Local_Control.6)EQU(Q2X.Command,17)BTD(Port_Data.Data_Transfer[0],0,Q2X.Write.Pulse_Freq.Far_Freq,24,8)BTD(Port_Data.Data_Transfer[1],0,Q2X.Write.Pulse_Freq.Far_Freq,16,8)BTD(Port_Data.Data_Transfer[2],0,Q2X.Write.Pulse_Freq.Far_Freq,8,8)BTD(Port_Data.Data_Transfer[3],0,Q2X.Write.Pulse_Freq.Far_Freq,0,8)BTD(Port_Data.Data_Transfer[4],0,Q2X.Write.Pulse_Freq.Near_Freq,24,8)BTD(Port_Data.Data_Transfer[5],0,Q2X.Write.Pulse_Freq.Near_Freq,16,8)BTD(Port_Data.Data_Transfer[6],0,Q2X.Write.Pulse_Freq.Near_Freq,8,8)BTD(Port_Data.Data_Transfer[7],0,Q2X.Write.Pulse_Freq.Near_Freq,0,8)OTU(Port_Data.Port_Read.[Port])OTL(Local_Control.6);
   55: NOP();
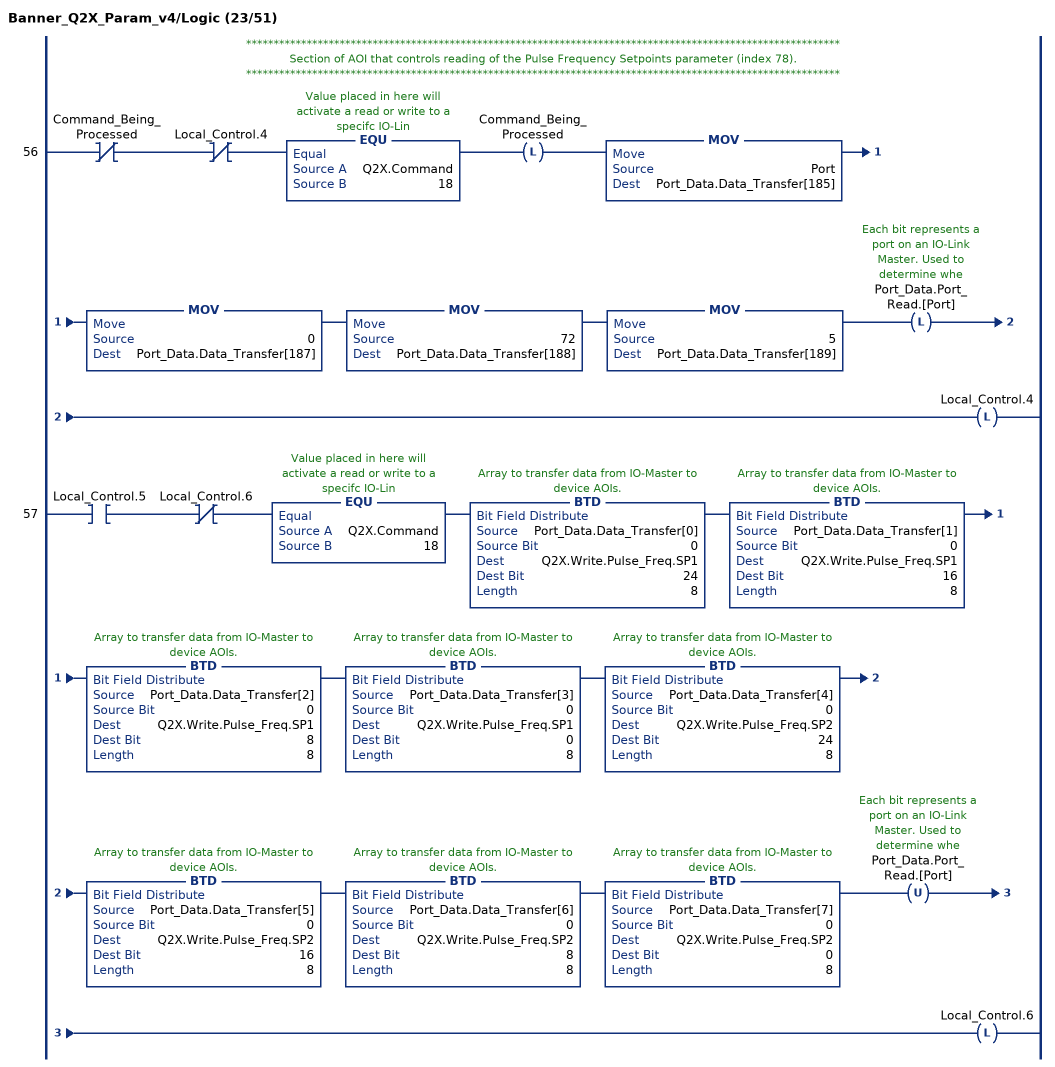
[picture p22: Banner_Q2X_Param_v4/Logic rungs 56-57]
   // ************************************************************************************************************
   // Section of AOI that controls reading of the Pulse Frequency Setpoints parameter (index 78).
   // ************************************************************************************************************
   56: XIO(Command_Being_Processed)XIO(Local_Control.4)EQU(Q2X.Command,18)OTL(Command_Being_Processed)MOV(Port,Port_Data.Data_Transfer[185])MOV(0,Port_Data.Data_Transfer[187])MOV(72,Port_Data.Data_Transfer[188])MOV(5,Port_Data.Data_Transfer[189])OTL(Port_Data.Port_Read.[Port])OTL(Local_Control.4);
   57: XIC(Local_Control.5)XIO(Local_Control.6)EQU(Q2X.Command,18)BTD(Port_Data.Data_Transfer[0],0,Q2X.Write.Pulse_Freq.SP1,24,8)BTD(Port_Data.Data_Transfer[1],0,Q2X.Write.Pulse_Freq.SP1,16,8)BTD(Port_Data.Data_Transfer[2],0,Q2X.Write.Pulse_Freq.SP1,8,8)BTD(Port_Data.Data_Transfer[3],0,Q2X.Write.Pulse_Freq.SP1,0,8)BTD(Port_Data.Data_Transfer[4],0,Q2X.Write.Pulse_Freq.SP2,24,8)BTD(Port_Data.Data_Transfer[5],0,Q2X.Write.Pulse_Freq.SP2,16,8)BTD(Port_Data.Data_Transfer[6],0,Q2X.Write.Pulse_Freq.SP2,8,8)BTD(Port_Data.Data_Transfer[7],0,Q2X.Write.Pulse_Freq.SP2,0,8)OTU(Port_Data.Port_Read.[Port])OTL(Local_Control.6);
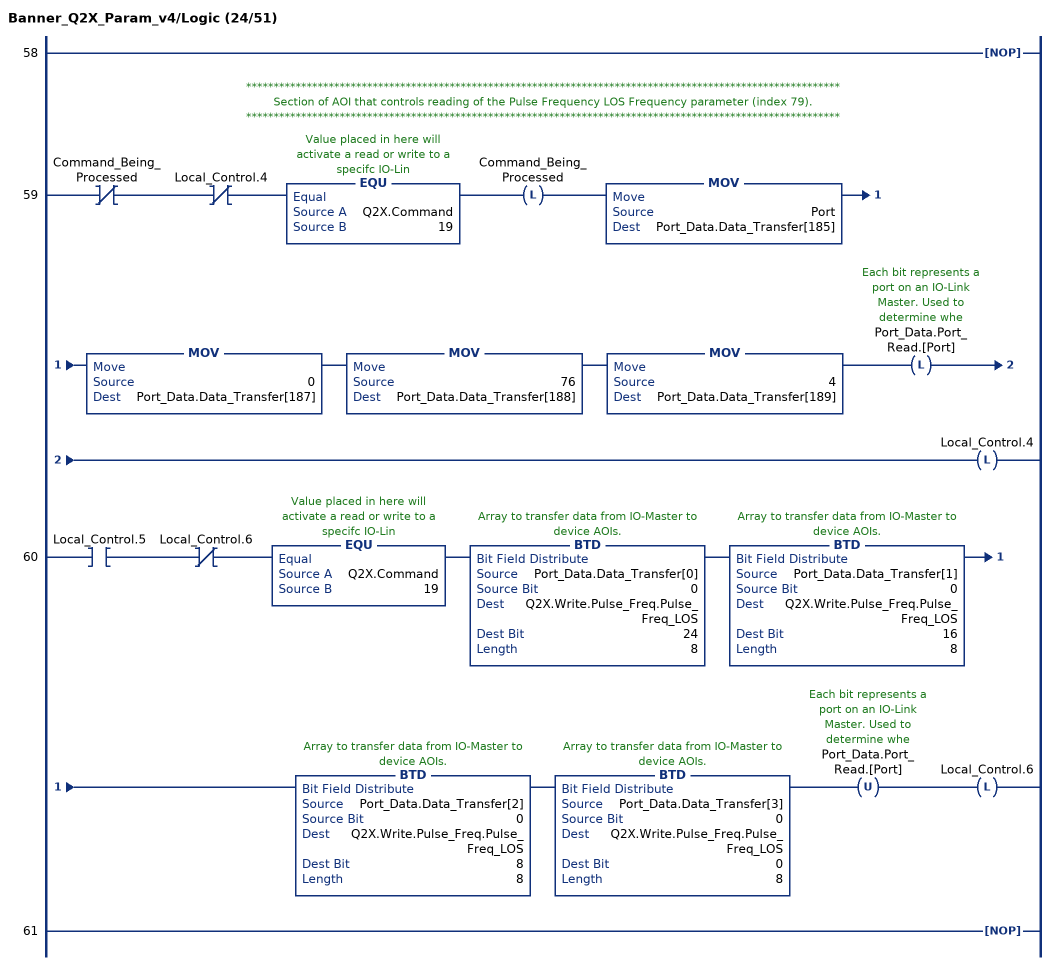
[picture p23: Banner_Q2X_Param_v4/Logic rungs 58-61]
   58: NOP();
   // ************************************************************************************************************
   // Section of AOI that controls reading of the Pulse Frequency LOS Frequency parameter (index 79).
   // ************************************************************************************************************
   59: XIO(Command_Being_Processed)XIO(Local_Control.4)EQU(Q2X.Command,19)OTL(Command_Being_Processed)MOV(Port,Port_Data.Data_Transfer[185])MOV(0,Port_Data.Data_Transfer[187])MOV(76,Port_Data.Data_Transfer[188])MOV(4,Port_Data.Data_Transfer[189])OTL(Port_Data.Port_Read.[Port])OTL(Local_Control.4);
   60: XIC(Local_Control.5)XIO(Local_Control.6)EQU(Q2X.Command,19)BTD(Port_Data.Data_Transfer[0],0,Q2X.Write.Pulse_Freq.Pulse_Freq_LOS,24,8)BTD(Port_Data.Data_Transfer[1],0,Q2X.Write.Pulse_Freq.Pulse_Freq_LOS,16,8)BTD(Port_Data.Data_Transfer[2],0,Q2X.Write.Pulse_Freq.Pulse_Freq_LOS,8,8)BTD(Port_Data.Data_Transfer[3],0,Q2X.Write.Pulse_Freq.Pulse_Freq_LOS,0,8)OTU(Port_Data.Port_Read.[Port])OTL(Local_Control.6);
   61: NOP();
